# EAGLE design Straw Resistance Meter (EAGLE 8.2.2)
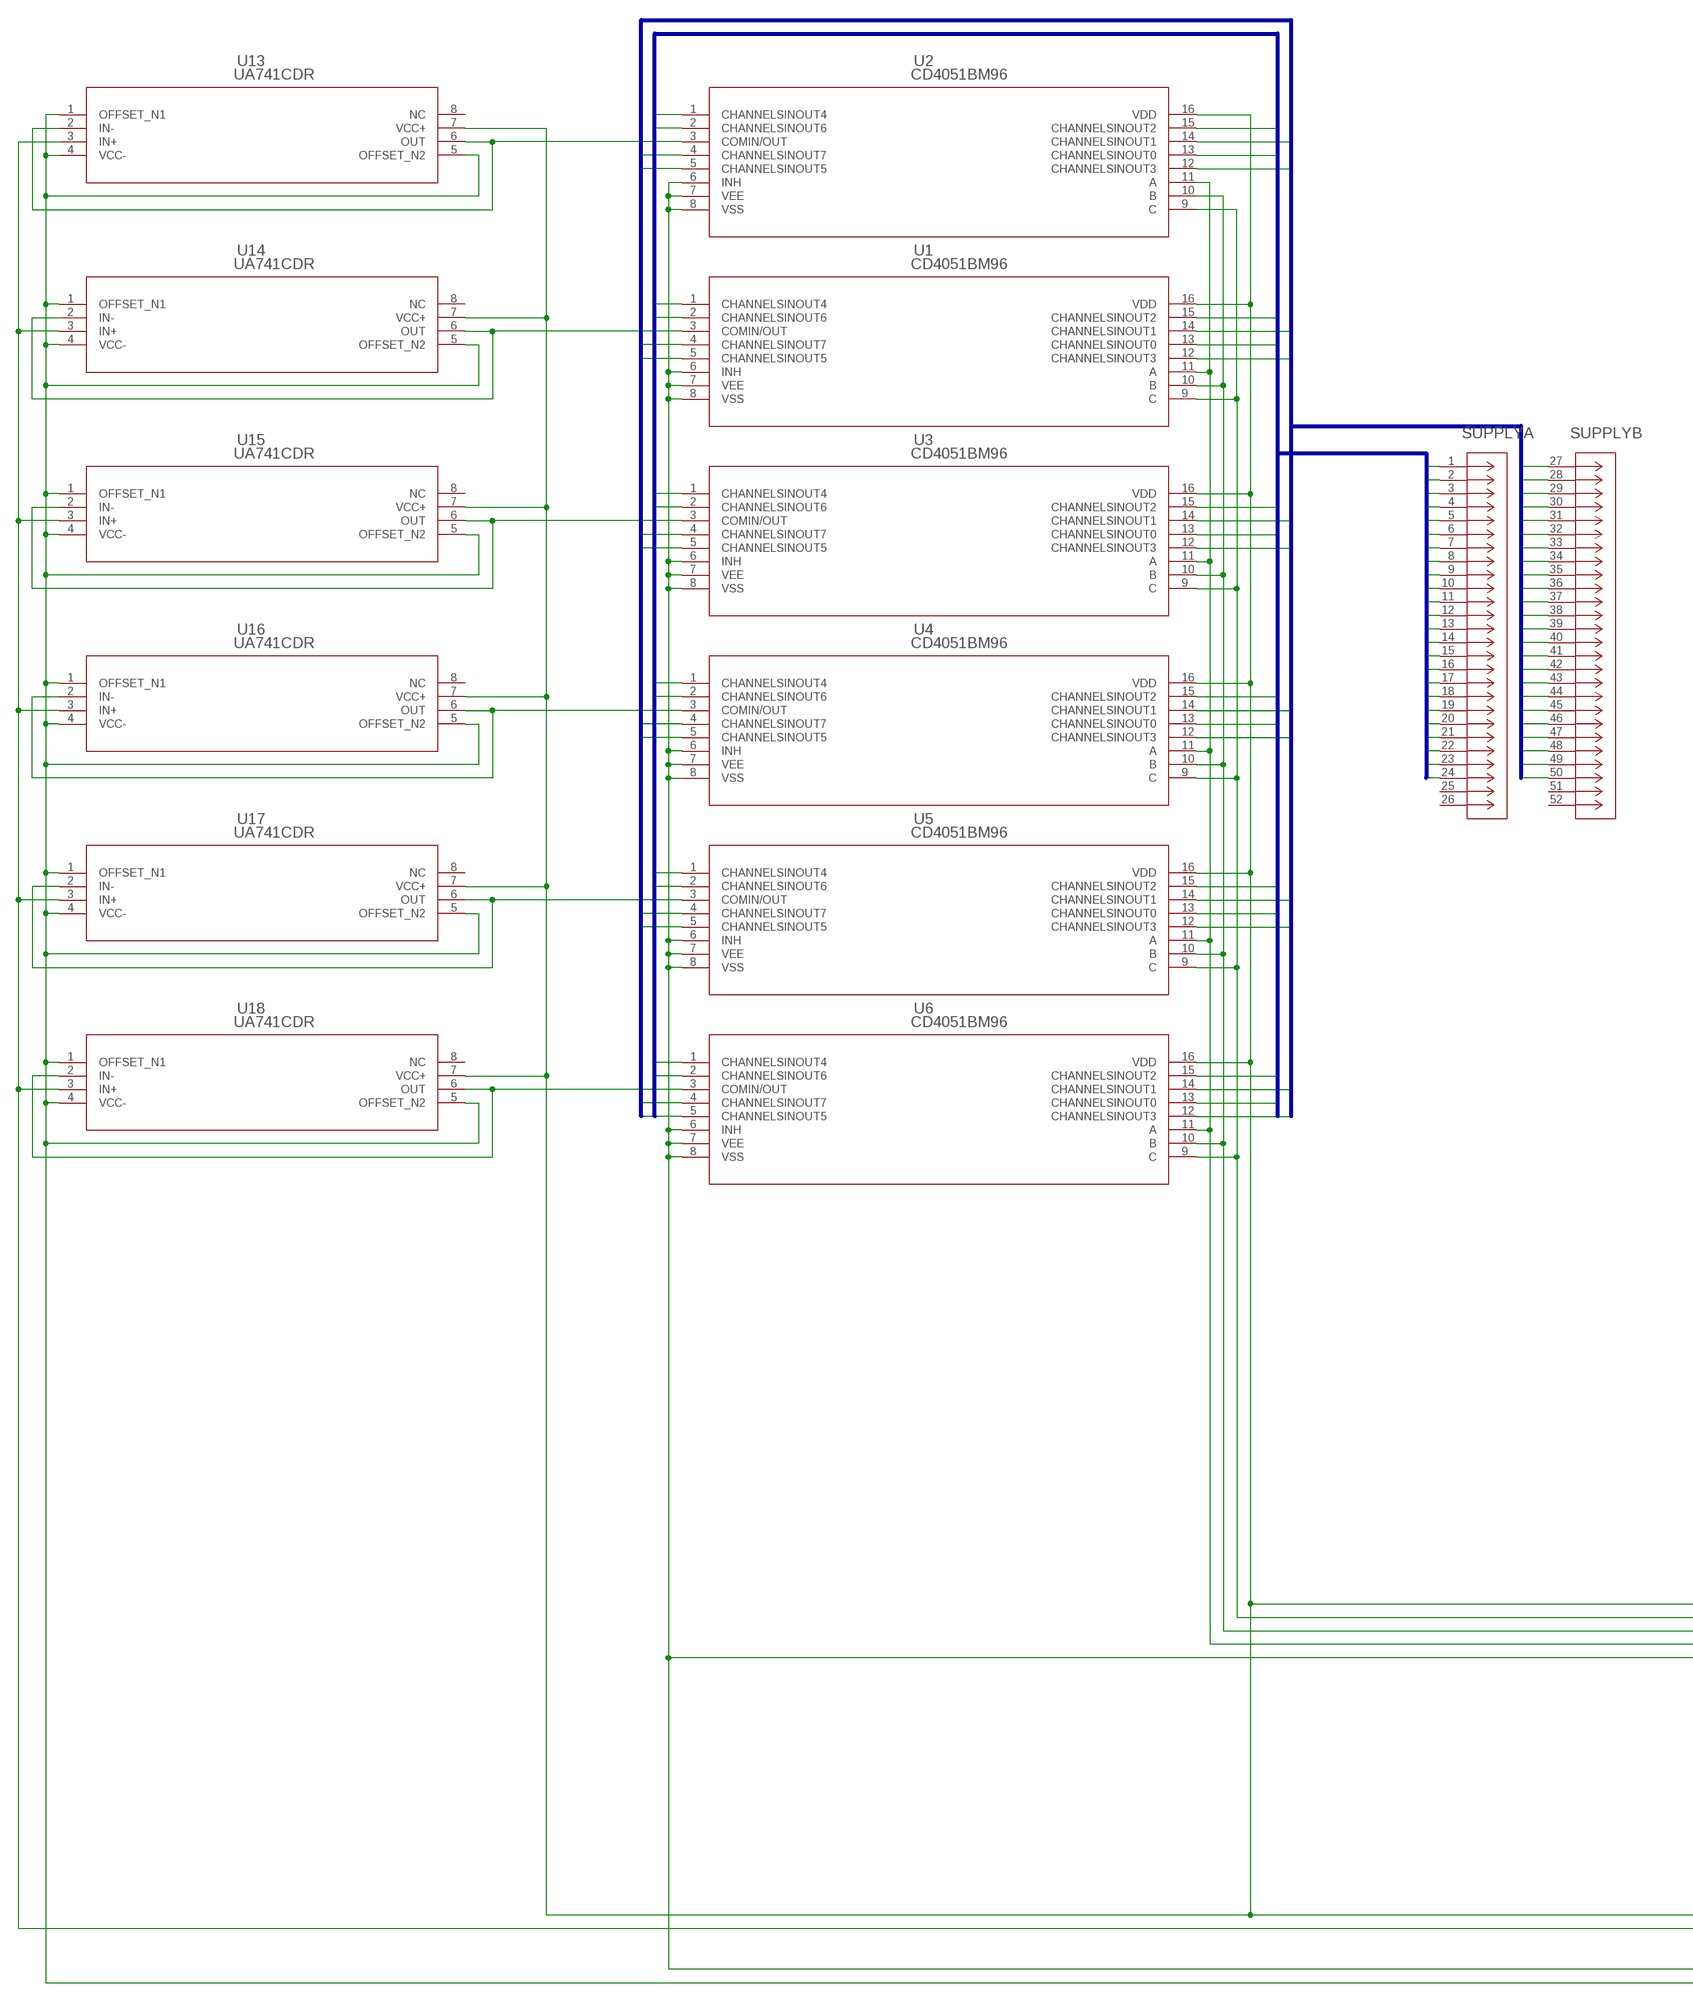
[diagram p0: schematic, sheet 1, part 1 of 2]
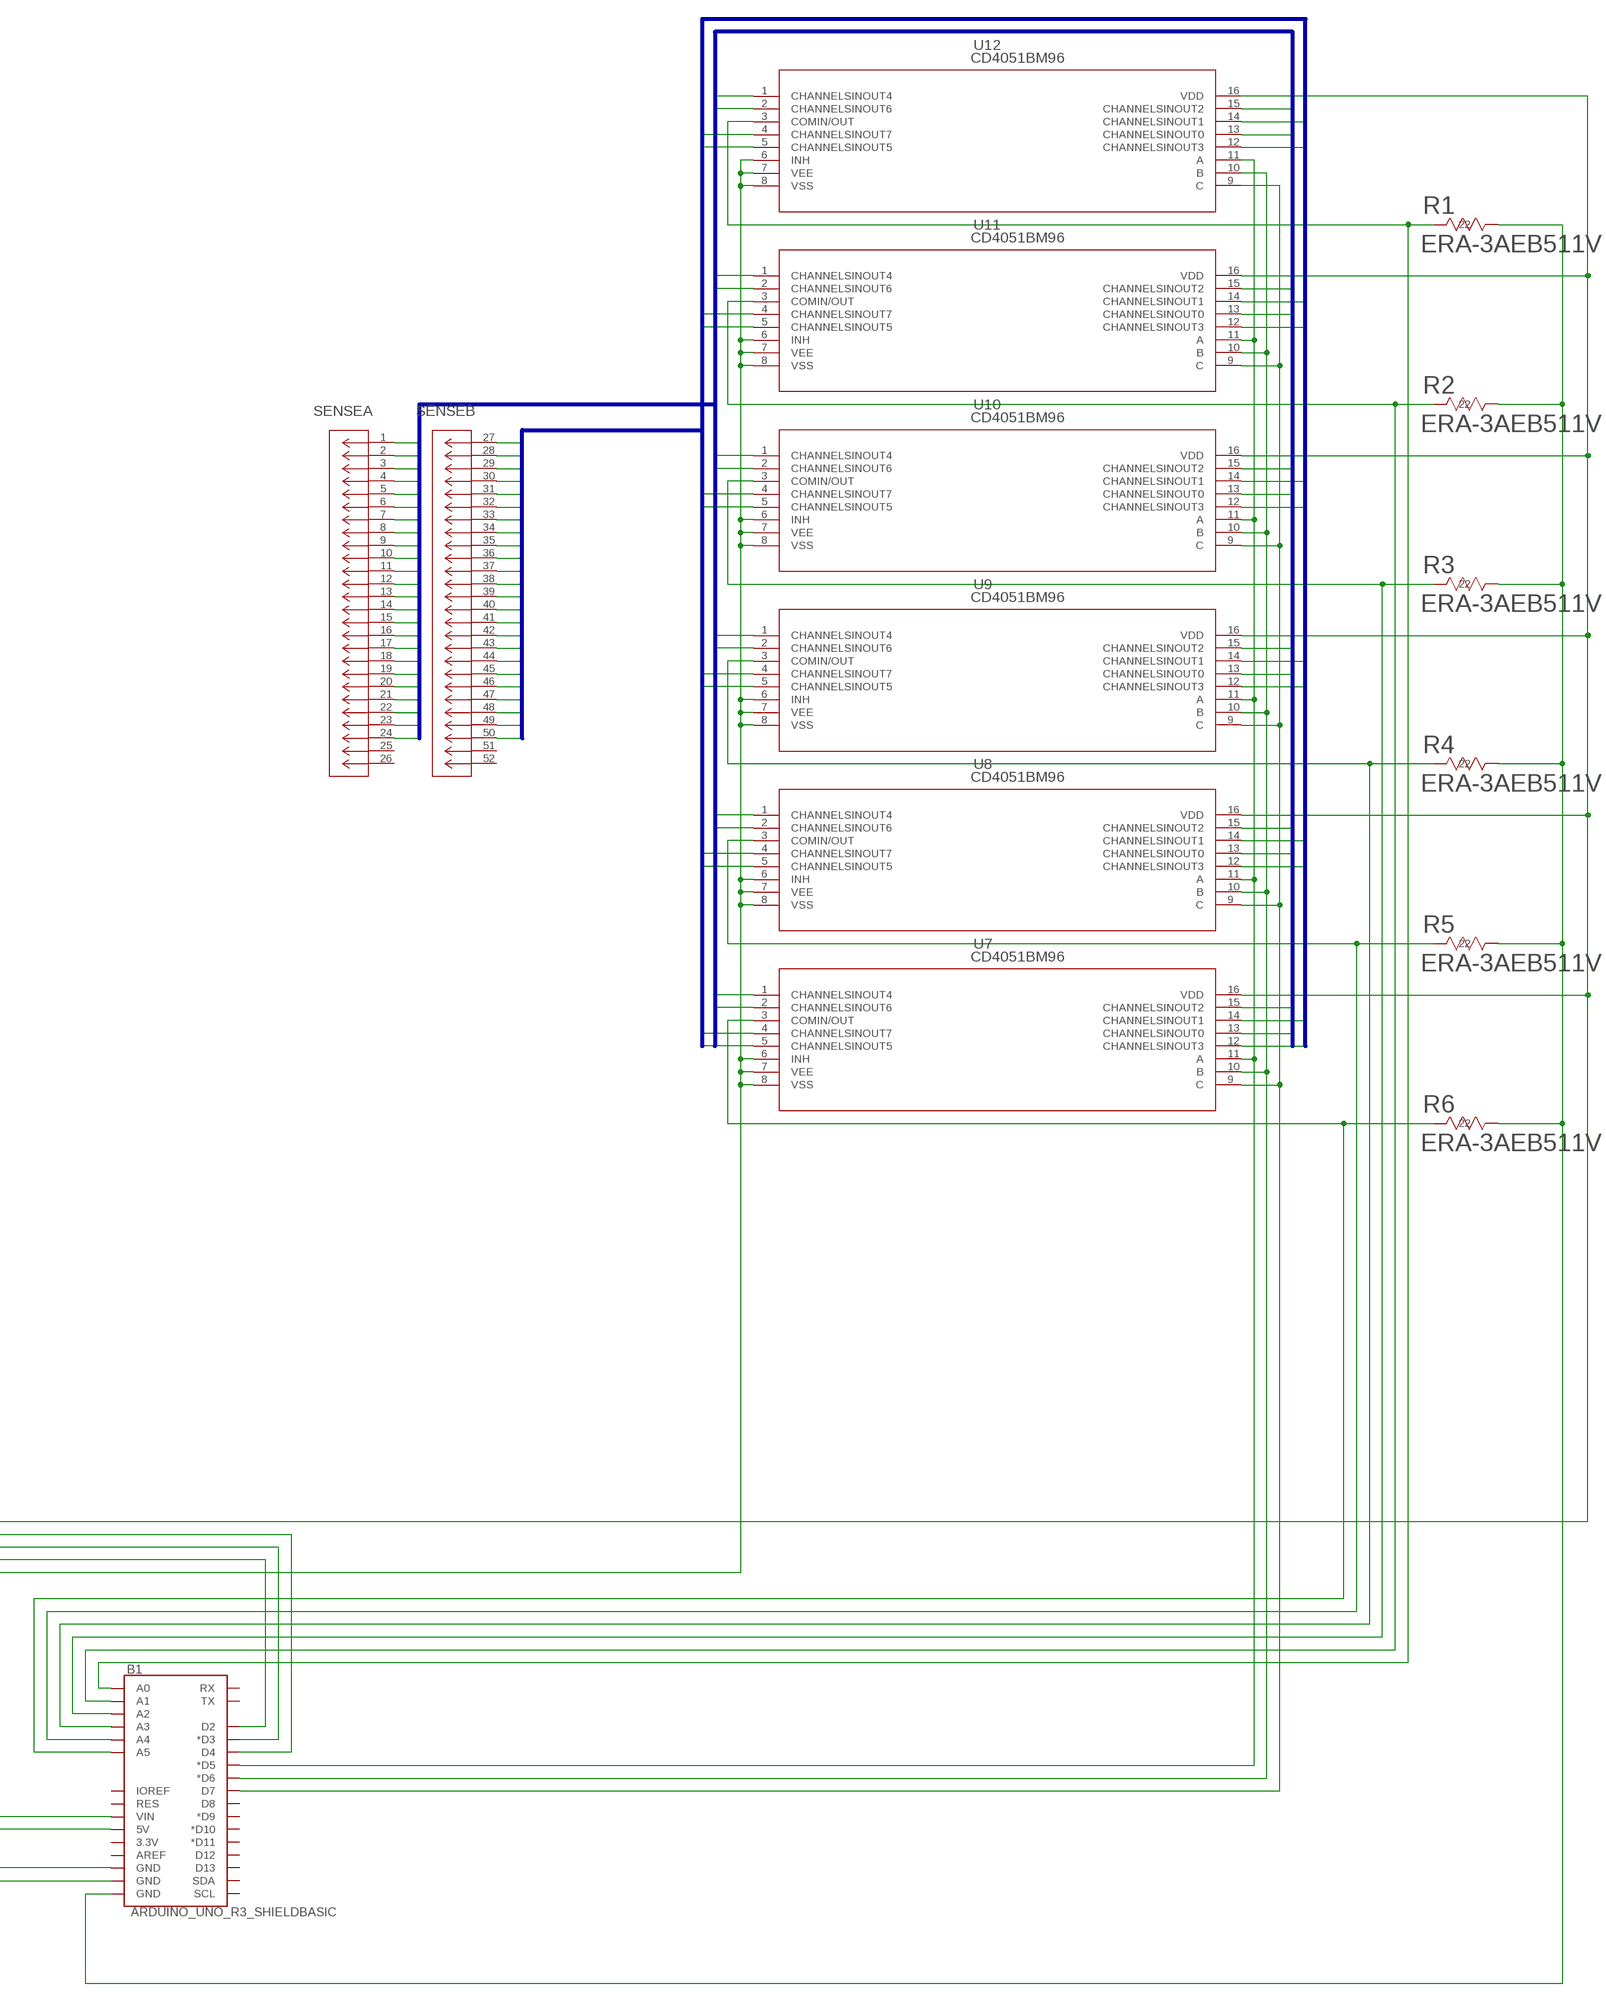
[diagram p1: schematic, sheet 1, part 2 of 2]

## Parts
B1  ARDUINO_UNO_R3_SHIELDBASIC  [UNO_R3_SHIELD]
R1  ERA-3AEB511V  [RC0603N]
R2  ERA-3AEB511V  [RC0603N]
R3  ERA-3AEB511V  [RC0603N]
R4  ERA-3AEB511V  [RC0603N]
R5  ERA-3AEB511V  [RC0603N]
R6  ERA-3AEB511V  [RC0603N]
SENSE  71918-150LF  [CON50_2X25_USZ_FCI]
SUPPLY  71918-150LF  [CON50_2X25_USZ_FCI]
U1  CD4051BM96  [D16]
U2  CD4051BM96  [D16]
U3  CD4051BM96  [D16]
U4  CD4051BM96  [D16]
U5  CD4051BM96  [D16]
U6  CD4051BM96  [D16]
U7  CD4051BM96  [D16]
U8  CD4051BM96  [D16]
U9  CD4051BM96  [D16]
U10  CD4051BM96  [D16]
U11  CD4051BM96  [D16]
U12  CD4051BM96  [D16]
U13  UA741CDR  [D8]
U14  UA741CDR  [D8]
U15  UA741CDR  [D8]
U16  UA741CDR  [D8]
U17  UA741CDR  [D8]
U18  UA741CDR  [D8]

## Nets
INNER_SENSE_BUS0: SENSE.1 U12.13(CHANNELSINOUT0)
INNER_SENSE_BUS1: SENSE.2 U12.15(CHANNELSINOUT2)
INNER_SENSE_BUS2: SENSE.3 U12.1(CHANNELSINOUT4)
INNER_SENSE_BUS3: SENSE.4 U12.2(CHANNELSINOUT6)
INNER_SENSE_BUS4: SENSE.5 U11.13(CHANNELSINOUT0)
INNER_SENSE_BUS5: SENSE.6 U11.15(CHANNELSINOUT2)
INNER_SENSE_BUS6: SENSE.7 U11.1(CHANNELSINOUT4)
INNER_SENSE_BUS7: SENSE.8 U11.2(CHANNELSINOUT6)
INNER_SENSE_BUS8: SENSE.9 U10.13(CHANNELSINOUT0)
INNER_SENSE_BUS9: SENSE.10 U10.15(CHANNELSINOUT2)
INNER_SENSE_BUS10: SENSE.11 U10.1(CHANNELSINOUT4)
INNER_SENSE_BUS11: SENSE.12 U10.2(CHANNELSINOUT6)
INNER_SENSE_BUS12: SENSE.13 U9.13(CHANNELSINOUT0)
INNER_SENSE_BUS13: SENSE.14 U9.15(CHANNELSINOUT2)
INNER_SENSE_BUS14: SENSE.15 U9.1(CHANNELSINOUT4)
INNER_SENSE_BUS15: SENSE.16 U9.2(CHANNELSINOUT6)
INNER_SENSE_BUS16: SENSE.17 U8.13(CHANNELSINOUT0)
INNER_SENSE_BUS17: SENSE.18 U8.15(CHANNELSINOUT2)
INNER_SENSE_BUS18: SENSE.19 U8.1(CHANNELSINOUT4)
INNER_SENSE_BUS19: SENSE.20 U8.2(CHANNELSINOUT6)
INNER_SENSE_BUS20: SENSE.21 U7.13(CHANNELSINOUT0)
INNER_SENSE_BUS21: SENSE.22 U7.15(CHANNELSINOUT2)
INNER_SENSE_BUS22: SENSE.23 U7.1(CHANNELSINOUT4)
INNER_SENSE_BUS23: SENSE.24 U7.2(CHANNELSINOUT6)
INNER_SUPPLY_BUS0: SUPPLY.1 U2.13(CHANNELSINOUT0)
INNER_SUPPLY_BUS1: SUPPLY.2 U2.15(CHANNELSINOUT2)
INNER_SUPPLY_BUS2: SUPPLY.3 U2.1(CHANNELSINOUT4)
INNER_SUPPLY_BUS3: SUPPLY.4 U2.2(CHANNELSINOUT6)
INNER_SUPPLY_BUS4: SUPPLY.5 U1.13(CHANNELSINOUT0)
INNER_SUPPLY_BUS5: SUPPLY.6 U1.15(CHANNELSINOUT2)
INNER_SUPPLY_BUS6: SUPPLY.7 U1.1(CHANNELSINOUT4)
INNER_SUPPLY_BUS7: SUPPLY.8 U1.2(CHANNELSINOUT6)
INNER_SUPPLY_BUS8: SUPPLY.9 U3.13(CHANNELSINOUT0)
INNER_SUPPLY_BUS9: SUPPLY.10 U3.15(CHANNELSINOUT2)
INNER_SUPPLY_BUS10: SUPPLY.11 U3.1(CHANNELSINOUT4)
INNER_SUPPLY_BUS11: SUPPLY.12 U3.2(CHANNELSINOUT6)
INNER_SUPPLY_BUS12: SUPPLY.13 U4.13(CHANNELSINOUT0)
INNER_SUPPLY_BUS13: SUPPLY.14 U4.15(CHANNELSINOUT2)
INNER_SUPPLY_BUS14: SUPPLY.15 U4.1(CHANNELSINOUT4)
INNER_SUPPLY_BUS15: SUPPLY.16 U4.2(CHANNELSINOUT6)
INNER_SUPPLY_BUS16: SUPPLY.17 U5.13(CHANNELSINOUT0)
INNER_SUPPLY_BUS17: SUPPLY.18 U5.15(CHANNELSINOUT2)
INNER_SUPPLY_BUS18: SUPPLY.19 U5.1(CHANNELSINOUT4)
INNER_SUPPLY_BUS19: SUPPLY.20 U5.2(CHANNELSINOUT6)
INNER_SUPPLY_BUS20: SUPPLY.21 U6.13(CHANNELSINOUT0)
INNER_SUPPLY_BUS21: SUPPLY.22 U6.15(CHANNELSINOUT2)
INNER_SUPPLY_BUS22: SUPPLY.23 U6.1(CHANNELSINOUT4)
INNER_SUPPLY_BUS23: SUPPLY.24 U6.2(CHANNELSINOUT6)
N$1 [Power]: B1.GND@2(GND) U1.6(INH) U1.7(VEE) U1.8(VSS) U2.6(INH) U2.7(VEE) U2.8(VSS) U3.6(INH) U3.7(VEE) U3.8(VSS) U4.6(INH) U4.7(VEE) U4.8(VSS) U5.6(INH) U5.7(VEE) U5.8(VSS) U6.6(INH) U6.7(VEE) U6.8(VSS) U7.6(INH) U7.7(VEE) U7.8(VSS) U8.6(INH) U8.7(VEE) U8.8(VSS) U9.6(INH) U9.7(VEE) U9.8(VSS) U10.6(INH) U10.7(VEE) U10.8(VSS) U11.6(INH) U11.7(VEE) U11.8(VSS) U12.6(INH) U12.7(VEE) U12.8(VSS)
N$2: U2.3(COMIN/OUT) U13.2(IN-) U13.6(OUT)
N$3 [Power]: B1.GND@1(GND) U13.1(OFFSET_N1) U13.4(VCC-) U13.5(OFFSET_N2) U14.1(OFFSET_N1) U14.4(VCC-) U14.5(OFFSET_N2) U15.1(OFFSET_N1) U15.4(VCC-) U15.5(OFFSET_N2) U16.1(OFFSET_N1) U16.4(VCC-) U16.5(OFFSET_N2) U17.1(OFFSET_N1) U17.4(VCC-) U17.5(OFFSET_N2) U18.1(OFFSET_N1) U18.4(VCC-) U18.5(OFFSET_N2)
N$4 [Power]: B1.VIN U1.16(VDD) U2.16(VDD) U3.16(VDD) U4.16(VDD) U5.16(VDD) U6.16(VDD) U7.16(VDD) U8.16(VDD) U9.16(VDD) U10.16(VDD) U11.16(VDD) U12.16(VDD) U13.7(VCC+) U14.7(VCC+) U15.7(VCC+) U16.7(VCC+) U17.7(VCC+) U18.7(VCC+)
N$5 [Power]: B1.5V U13.3(IN+) U14.3(IN+) U15.3(IN+) U16.3(IN+) U17.3(IN+) U18.3(IN+)
N$6: B1.D4 U1.9(C) U2.9(C) U3.9(C) U4.9(C) U5.9(C) U6.9(C)
N$7: U1.3(COMIN/OUT) U14.2(IN-) U14.6(OUT)
N$8: B1.D3(*D3) U1.10(B) U2.10(B) U3.10(B) U4.10(B) U5.10(B) U6.10(B)
N$9: B1.D2 U1.11(A) U2.11(A) U3.11(A) U4.11(A) U5.11(A) U6.11(A)
N$10: U3.3(COMIN/OUT) U15.2(IN-) U15.6(OUT)
N$11: B1.D5(*D5) U7.11(A) U8.11(A) U9.11(A) U10.11(A) U11.11(A) U12.11(A)
N$12: B1.D6(*D6) U7.10(B) U8.10(B) U9.10(B) U10.10(B) U11.10(B) U12.10(B)
N$13: U4.3(COMIN/OUT) U16.2(IN-) U16.6(OUT)
N$14: B1.D7 U7.9(C) U8.9(C) U9.9(C) U10.9(C) U11.9(C) U12.9(C)
N$15: B1.A0 R1.2 U12.3(COMIN/OUT)
N$16: U5.3(COMIN/OUT) U17.2(IN-) U17.6(OUT)
N$17: B1.A1 R2.2 U11.3(COMIN/OUT)
N$18: B1.A3 R4.2 U9.3(COMIN/OUT)
N$19: U6.3(COMIN/OUT) U18.2(IN-) U18.6(OUT)
N$20: B1.A4 R5.2 U8.3(COMIN/OUT)
N$21 [Power]: B1.GND@0(GND) R1.1 R2.1 R3.1 R4.1 R5.1 R6.1
N$22: B1.A5 R6.2 U7.3(COMIN/OUT)
N$23: B1.A2 R3.2 U10.3(COMIN/OUT)
OUTER_SENSE_BUS0: SENSE.27 U12.14(CHANNELSINOUT1)
OUTER_SENSE_BUS1: SENSE.28 U12.12(CHANNELSINOUT3)
OUTER_SENSE_BUS2: SENSE.29 U12.5(CHANNELSINOUT5)
OUTER_SENSE_BUS3: SENSE.30 U12.4(CHANNELSINOUT7)
OUTER_SENSE_BUS4: SENSE.31 U11.14(CHANNELSINOUT1)
OUTER_SENSE_BUS5: SENSE.32 U11.12(CHANNELSINOUT3)
OUTER_SENSE_BUS6: SENSE.33 U11.5(CHANNELSINOUT5)
OUTER_SENSE_BUS7: SENSE.34 U11.4(CHANNELSINOUT7)
OUTER_SENSE_BUS8: SENSE.35 U10.14(CHANNELSINOUT1)
OUTER_SENSE_BUS9: SENSE.36 U10.12(CHANNELSINOUT3)
OUTER_SENSE_BUS10: SENSE.37 U10.5(CHANNELSINOUT5)
OUTER_SENSE_BUS11: SENSE.38 U10.4(CHANNELSINOUT7)
OUTER_SENSE_BUS12: SENSE.39 U9.14(CHANNELSINOUT1)
OUTER_SENSE_BUS13: SENSE.40 U9.12(CHANNELSINOUT3)
OUTER_SENSE_BUS14: SENSE.41 U9.5(CHANNELSINOUT5)
OUTER_SENSE_BUS15: SENSE.42 U9.4(CHANNELSINOUT7)
OUTER_SENSE_BUS16: SENSE.43 U8.14(CHANNELSINOUT1)
OUTER_SENSE_BUS17: SENSE.44 U8.12(CHANNELSINOUT3)
OUTER_SENSE_BUS18: SENSE.45 U8.5(CHANNELSINOUT5)
OUTER_SENSE_BUS19: SENSE.46 U8.4(CHANNELSINOUT7)
OUTER_SENSE_BUS20: SENSE.47 U7.14(CHANNELSINOUT1)
OUTER_SENSE_BUS21: SENSE.48 U7.12(CHANNELSINOUT3)
OUTER_SENSE_BUS22: SENSE.49 U7.5(CHANNELSINOUT5)
OUTER_SENSE_BUS23: SENSE.50 U7.4(CHANNELSINOUT7)
OUTER_SUPPLY_BUS0: SUPPLY.27 U2.14(CHANNELSINOUT1)
OUTER_SUPPLY_BUS1: SUPPLY.28 U2.12(CHANNELSINOUT3)
OUTER_SUPPLY_BUS2: SUPPLY.29 U2.5(CHANNELSINOUT5)
OUTER_SUPPLY_BUS3: SUPPLY.30 U2.4(CHANNELSINOUT7)
OUTER_SUPPLY_BUS4: SUPPLY.31 U1.14(CHANNELSINOUT1)
OUTER_SUPPLY_BUS5: SUPPLY.32 U1.12(CHANNELSINOUT3)
OUTER_SUPPLY_BUS6: SUPPLY.33 U1.5(CHANNELSINOUT5)
OUTER_SUPPLY_BUS7: SUPPLY.34 U1.4(CHANNELSINOUT7)
OUTER_SUPPLY_BUS8: SUPPLY.35 U3.14(CHANNELSINOUT1)
OUTER_SUPPLY_BUS9: SUPPLY.36 U3.12(CHANNELSINOUT3)
OUTER_SUPPLY_BUS10: SUPPLY.37 U3.5(CHANNELSINOUT5)
OUTER_SUPPLY_BUS11: SUPPLY.38 U3.4(CHANNELSINOUT7)
OUTER_SUPPLY_BUS12: SUPPLY.39 U4.14(CHANNELSINOUT1)
OUTER_SUPPLY_BUS13: SUPPLY.40 U4.12(CHANNELSINOUT3)
OUTER_SUPPLY_BUS14: SUPPLY.41 U4.5(CHANNELSINOUT5)
OUTER_SUPPLY_BUS15: SUPPLY.42 U4.4(CHANNELSINOUT7)
OUTER_SUPPLY_BUS16: SUPPLY.43 U5.14(CHANNELSINOUT1)
OUTER_SUPPLY_BUS17: SUPPLY.44 U5.12(CHANNELSINOUT3)
OUTER_SUPPLY_BUS18: SUPPLY.45 U5.5(CHANNELSINOUT5)
OUTER_SUPPLY_BUS19: SUPPLY.46 U5.4(CHANNELSINOUT7)
OUTER_SUPPLY_BUS20: SUPPLY.47 U6.14(CHANNELSINOUT1)
OUTER_SUPPLY_BUS21: SUPPLY.48 U6.12(CHANNELSINOUT3)
OUTER_SUPPLY_BUS22: SUPPLY.49 U6.5(CHANNELSINOUT5)
OUTER_SUPPLY_BUS23: SUPPLY.50 U6.4(CHANNELSINOUT7)
Unconnected: B1.3.3V B1.AREF B1.D8 B1.D9(*D9) B1.D10(*D10) B1.D11(*D11) B1.D12 B1.D13 B1.IOREF B1.RES B1.RX B1.SCL B1.SDA B1.TX SENSE.25 SENSE.26 SENSE.51 SENSE.52 SUPPLY.25 SUPPLY.26 SUPPLY.51 SUPPLY.52 U13.8(NC) U14.8(NC) U15.8(NC) U16.8(NC) U17.8(NC) U18.8(NC)

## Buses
INNER_SUPPLY_BUS[0..23]
OUTER_SUPPLY_BUS[0..23]
INNER_SENSE_BUS[0..23]
OUTER_SENSE_BUS[0..23]

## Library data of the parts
B1 = SparkFun-Boards:ARDUINO_UNO_R3_SHIELD: Arduino R3 Shield Footprint Shield form compatible with the Arduino Uno R3. SparkFun Products: MG2639 Cellular Shield MIDI Shield R3 Stackable Headers Kit
R1-R6 = P510DBCT-ND:ERA-3AEB511V; MANUFACTURER_PART_NUMBER: ERA3AEB511V; VENDOR: Panasonic
SENSE SUPPLY = 609-1759-ND:71918-150LF; MANUFACTURER_PART_NUMBER: 71918150LF; VENDOR: FCI
U1-U12 = 296-14271-1-ND:CD4051BM96; MANUFACTURER_PART_NUMBER: CD4051BM96; VENDOR: Texas Instruments
U13-U18 = opamp_ti:UA741CDR; MANUFACTURER_PART_NUMBER: UA741CDR; VENDOR: Texas Instruments

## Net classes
0 default: width 0.254 mm, drill 0.3 mm, clearance 0.152 mm
1 Power: width 0.61 mm, drill 0.3 mm, clearance 0.152 mm

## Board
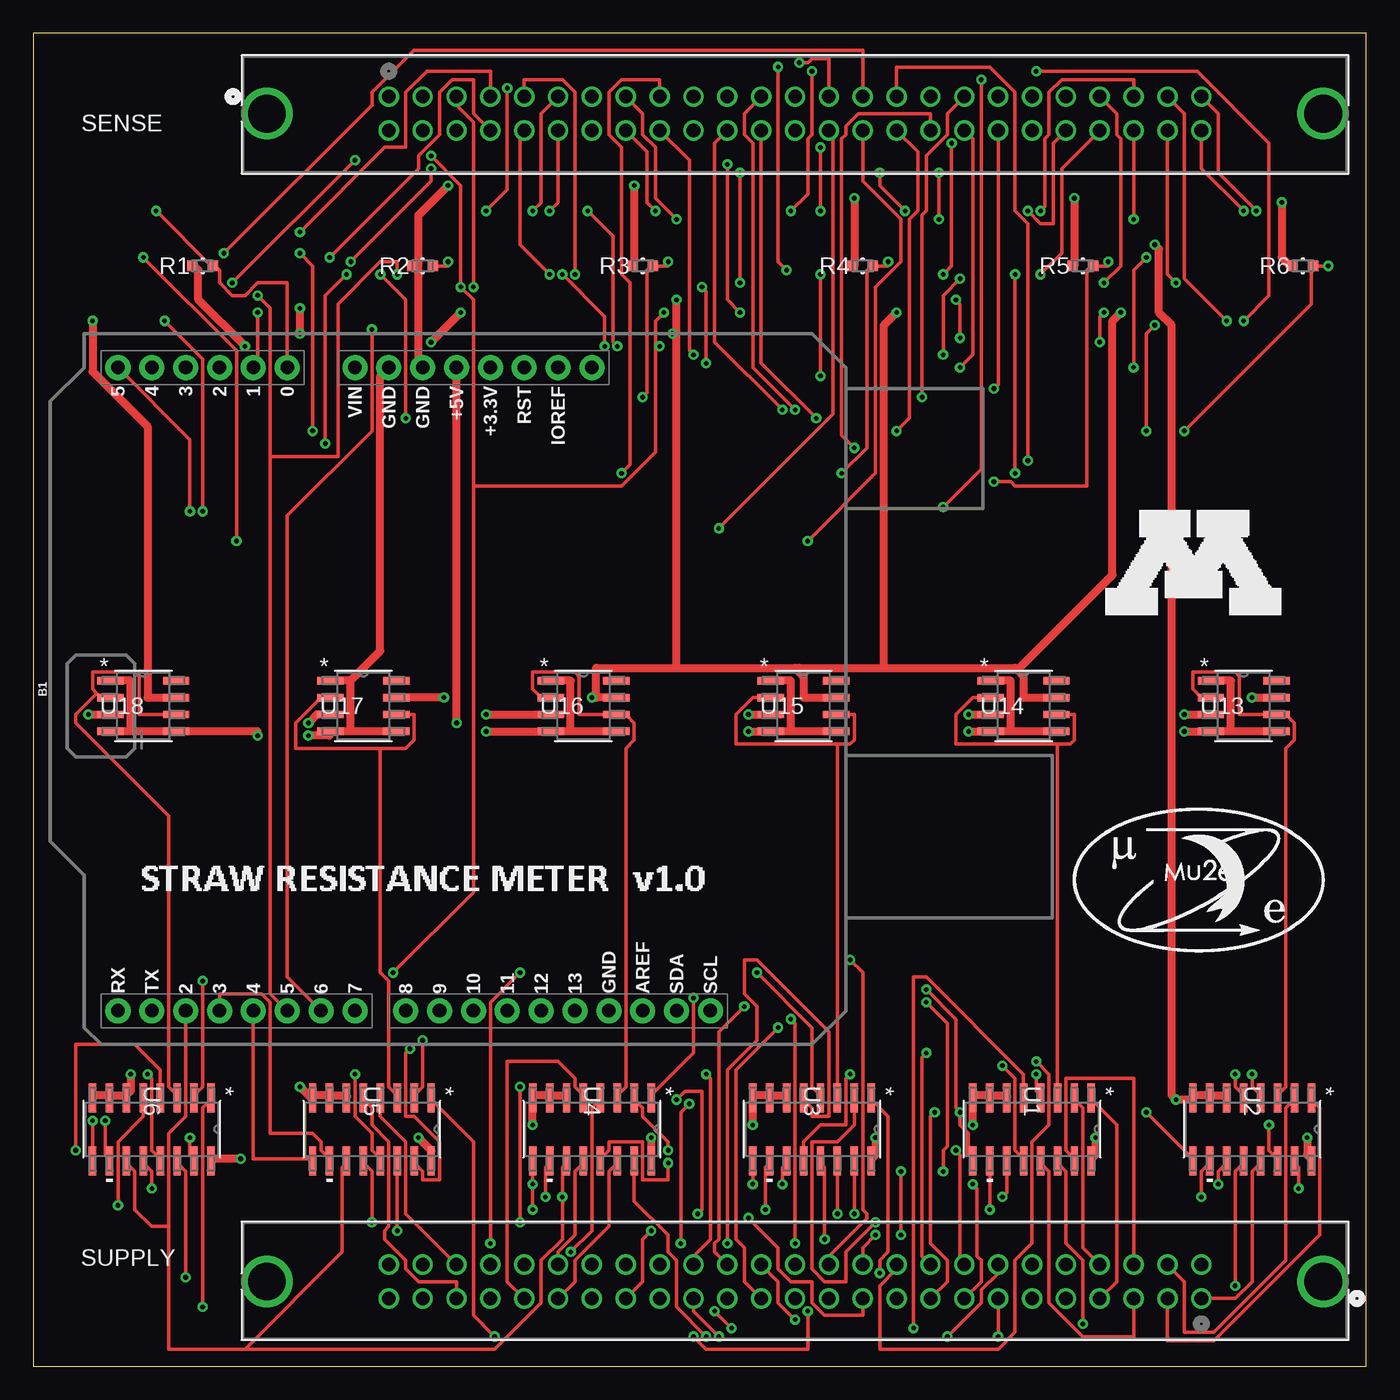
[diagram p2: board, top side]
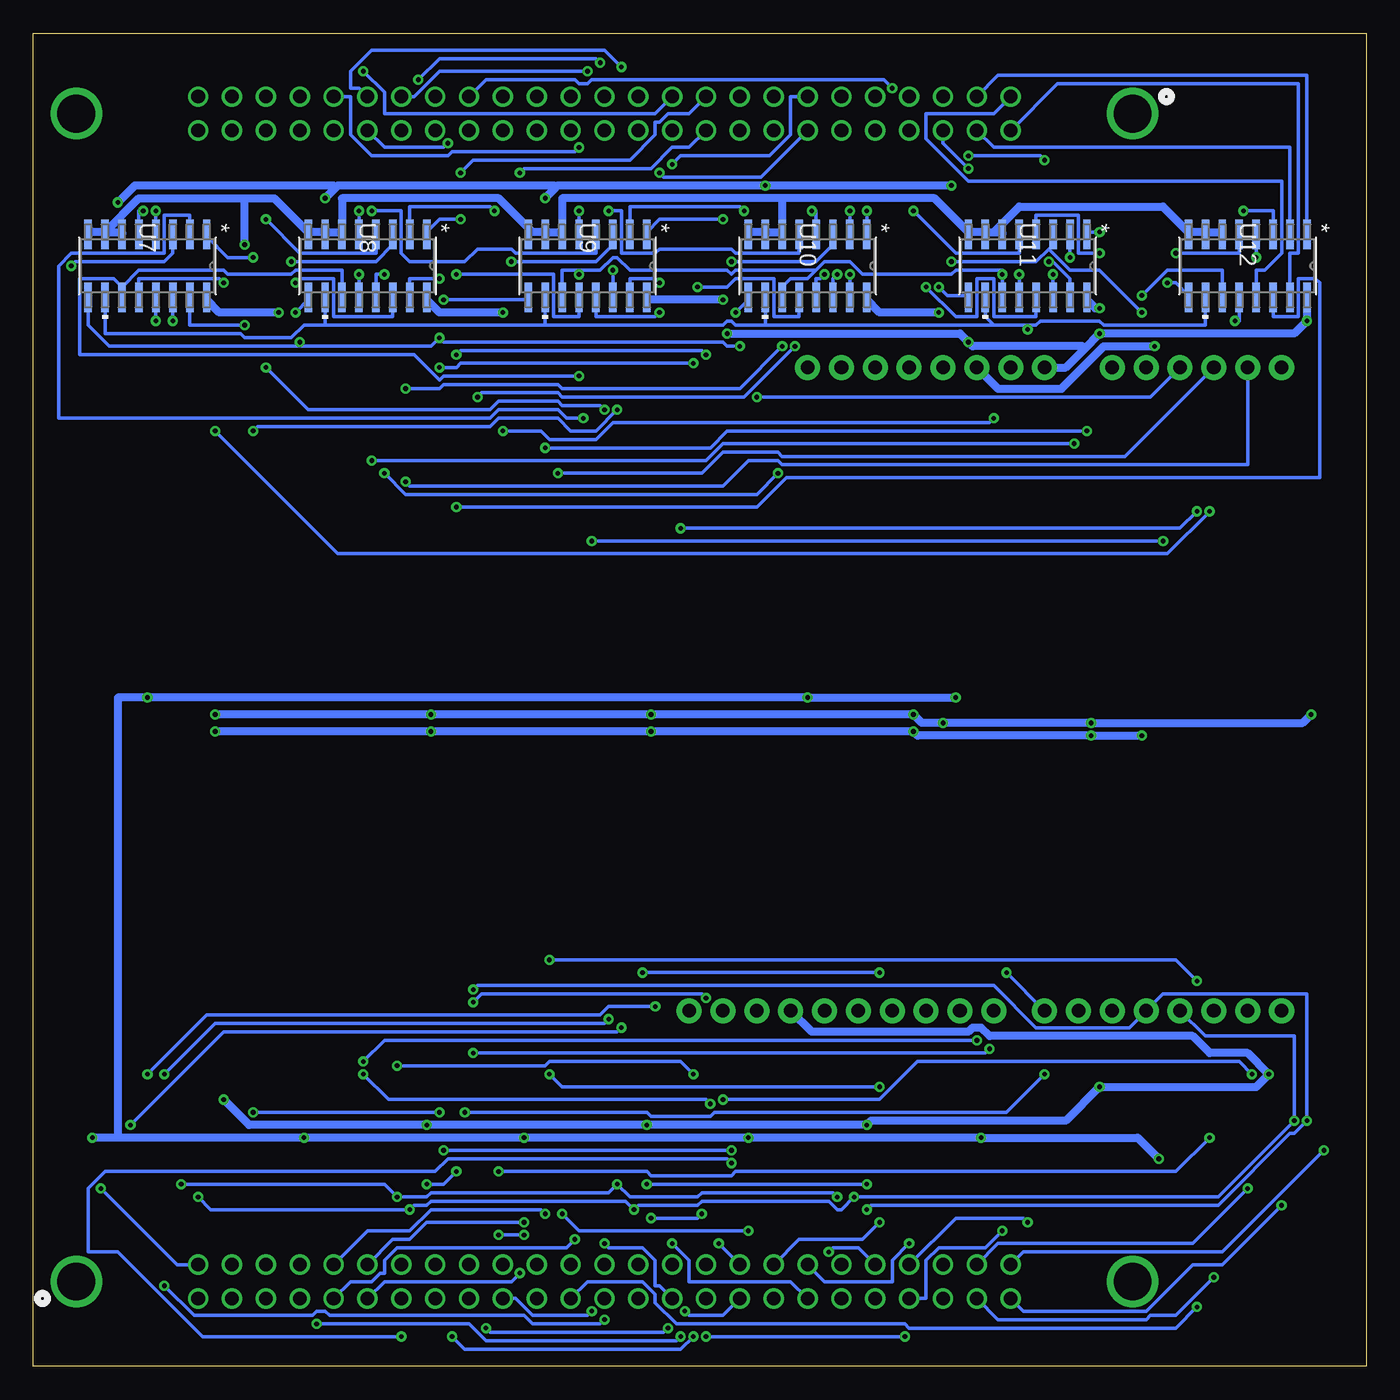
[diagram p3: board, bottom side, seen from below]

Size 100 x 100 mm. Coordinates in mm from the lower left corner, seen from the top.
Outline: 0,0 100,0 100,100 0,100 0,0
Copper layers (1*16): Top 0.035mm / dielectric 1.5mm / Bottom 0.035mm
Design rules "default": minimum track width 6mil, minimum drill 0.35mm, track to track 6mil, track to pad 6mil, pad to pad 6mil, via to via 6mil, smd to smd 6mil, copper to edge 40mil, drill to drill 6mil, minimum pad ring 10mil, minimum via ring 8mil, stop-mask expansion 4mil, vias tented up to drill 0mil, thermal gap 10mil

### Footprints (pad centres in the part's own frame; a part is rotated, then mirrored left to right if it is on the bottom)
UNO_R3_SHIELD = drill 1.016 pad 1.88: 3.3V 24.13,-2.54; 5V 24.13,0; A0 24.13,12.7; A1 24.13,15.24; A2 24.13,17.78; A3 24.13,20.32; A4 24.13,22.86; A5 24.13,25.4; AREF -24.13,-13.97; D2 -24.13,20.32; D3 -24.13,17.78; D4 -24.13,15.24; D5 -24.13,12.7; D6 -24.13,10.16; D7 -24.13,7.62; D8 -24.13,3.81; D9 -24.13,1.27; D10 -24.13,-1.27; D11 -24.13,-3.81; D12 -24.13,-6.35; D13 -24.13,-8.89; GND@0 24.13,2.54; GND@1 24.13,5.08; GND@2 -24.13,-11.43; IOREF 24.13,-7.62; NC 24.13,-10.16; RES 24.13,-5.08; RX -24.13,25.4; SCL -24.13,-19.05; SDA -24.13,-16.51; TX -24.13,22.86; VIN 24.13,7.62
RC0603N = smd 0.756 x 0.8: 1 -0.778,0; 2 0.778,0
CON50_2X25_USZ_FCI = drill 1.016 pad 1.524: 1 -60.96,2.54; 2 -60.96,0; 3 -58.42,2.54; 4 -58.42,0; 5 -55.88,2.54; 6 -55.88,0; 7 -53.34,2.54; 8 -53.34,0; 9 -50.8,2.54; 10 -50.8,0; 11 -48.26,2.54; 12 -48.26,0; 13 -45.72,2.54; 14 -45.72,0; 15 -43.18,2.54; 16 -43.18,0; 17 -40.64,2.54; 18 -40.64,0; 19 -38.1,2.54; 20 -38.1,0; 21 -35.56,2.54; 22 -35.56,0; 23 -33.02,2.54; 24 -33.02,0; 25 -30.48,2.54; 26 -30.48,0; 27 -27.94,2.54; 28 -27.94,0; 29 -25.4,2.54; 30 -25.4,0; 31 -22.86,2.54; 32 -22.86,0; 33 -20.32,2.54; 34 -20.32,0; 35 -17.78,2.54; 36 -17.78,0; 37 -15.24,2.54; 38 -15.24,0; 39 -12.7,2.54; 40 -12.7,0; 41 -10.16,2.54; 42 -10.16,0; 43 -7.62,2.54; 44 -7.62,0; 45 -5.08,2.54; 46 -5.08,0; 47 -2.54,2.54; 48 -2.54,0; 49 0,2.54; 50 0,0 | drill 2.845 pad 3.353: 51 -70.104,1.27; 52 9.144,1.27
D16 = smd 2.184 x 0.559: 1 -2.362,4.445; 2 -2.362,3.175; 3 -2.362,1.905; 4 -2.362,0.635; 5 -2.362,-0.635; 6 -2.362,-1.905; 7 -2.362,-3.175; 8 -2.362,-4.445; 9 2.362,-4.445; 10 2.362,-3.175; 11 2.362,-1.905; 12 2.362,-0.635; 13 2.362,0.635; 14 2.362,1.905; 15 2.362,3.175; 16 2.362,4.445
D8 = smd 1.981 x 0.559: 1 -2.464,1.905; 2 -2.464,0.635; 3 -2.464,-0.635; 4 -2.464,-1.905; 5 2.464,-1.905; 6 2.464,-0.635; 7 2.464,0.635; 8 2.464,1.905

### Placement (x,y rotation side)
B1  31.75,50.8 90 top
R1  12.7,82.55 0 top
R2  29.21,82.55 0 top
R3  45.72,82.55 0 top
R4  62.23,82.55 0 top
R5  78.74,82.55 0 top
R6  95.25,82.55 0 top
SENSE  87.63,92.71 0 top
SUPPLY  26.67,7.62 180 top
U1  74.93,17.78 270 top
U2  91.44,17.78 270 top
U3  58.42,17.78 270 top
U4  41.91,17.78 270 top
U5  25.4,17.78 270 top
U6  8.89,17.78 270 top
U7  91.44,82.55 270 bottom
U8  74.93,82.55 270 bottom
U9  58.42,82.55 270 bottom
U10  41.91,82.55 270 bottom
U11  25.4,82.55 270 bottom
U12  8.89,82.55 270 bottom
U13  90.81,49.53 0 top
U14  74.3,49.53 0 top
U15  57.78,49.53 0 top
U16  41.27,49.53 0 top
U17  24.77,49.53 0 top
U18  8.26,49.53 0 top

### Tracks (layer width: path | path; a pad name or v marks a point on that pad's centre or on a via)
INNER_SENSE_BUS0
  Bottom 0.254: U12.13 8.26,82.23 7.62,82.23 6.35,83.5 6.35,88.9 29.84,88.9 33.02,92.08 33.02,93.98 27.94,93.98 SENSE.1
INNER_SENSE_BUS1
  Bottom 0.254: U12.15 5.71,83.5 5.08,83.5 5.08,96.2 23.18,96.2 SENSE.2
INNER_SENSE_BUS2
  Bottom 0.254: U12.1 4.45,96.84 27.62,96.84 SENSE.3
INNER_SENSE_BUS3
  Bottom 0.254: U12.2 5.71,91.44 27.94,91.44 SENSE.4
INNER_SENSE_BUS4  (via drill 0.35)
  Top 0.254: v33.02,80.96 33.02,93.34 31.75,94.61 SENSE.5
  Bottom 0.254: U11.13 24.77,78.74 27.94,78.74 27.94,81.6 29.21,81.6 29.21,78.74 30.8,78.74 v33.02,80.96
INNER_SENSE_BUS5  (via drill 0.35)
  Top 0.254: v23.81,82.87 29.84,88.9 v29.84,89.85
  Bottom 0.254: U11.15 22.23,81.6 23.5,82.87 v23.81,82.87 | v29.84,89.85 31.75,91.76 SENSE.6
INNER_SENSE_BUS6  (via drill 0.35)
  Top 0.254: v20,85.09 26.35,91.44 27.94,91.44 27.94,95.57 29.53,97.16 34.29,97.16 SENSE.7
  Bottom 0.254: v20,85.09 20.95,85.09 U11.1
INNER_SENSE_BUS7  (via drill 0.35)
  Top 0.254: v22.23,83.19 28.89,89.85 28.89,90.81 30.48,92.39 30.48,95.57 31.43,96.52 33.02,96.52 33.02,93.98 SENSE.8
  Bottom 0.254: v22.23,83.19 U11.2
INNER_SENSE_BUS8  (via drill 0.35)
  Top 0.254: v40.64,81.92 40.64,95.57 39.69,96.52 36.83,96.52 SENSE.9
  Bottom 0.254: U10.13 41.27,81.6 40.96,81.6 v40.64,81.92
INNER_SENSE_BUS9  (via drill 0.35)
  Top 0.254: v38.73,81.92 36.51,84.14 36.51,92.39 SENSE.10
  Bottom 0.254: v38.73,81.92 U10.15
INNER_SENSE_BUS10  (via drill 0.35)
  Top 0.254: v37.47,86.68 38.1,87.31 38.1,93.98 SENSE.11
  Bottom 0.254: v37.47,86.68 U10.1
INNER_SENSE_BUS11  (via drill 0.35)
  Top 0.254: v38.73,86.68 39.37,87.31 SENSE.12
  Bottom 0.254: v38.73,86.68 U10.2
INNER_SENSE_BUS12  (via drill 0.35)
  Top 0.254: v53.02,79.06 52.07,80.01 v52.07,90.17
  Bottom 0.254: U9.13 57.78,78.74 53.34,78.74 v53.02,79.06 | v52.07,90.17 51.44,90.81 44.77,90.81 43.18,92.39 43.18,95.25 SENSE.13
INNER_SENSE_BUS13  (via drill 0.35)
  Top 0.254: v53.02,89.53 v53.02,81.28
  Bottom 0.254: U9.15 55.24,81.6 53.34,81.6 v53.02,81.28 | v53.02,89.53 52.7,89.22 45.4,89.22 SENSE.14
INNER_SENSE_BUS14  (via drill 0.35)
  Top 0.254: v48.26,86.04 46.67,87.63 46.67,91.44 45.72,92.39 45.72,93.98 SENSE.15
  Bottom 0.254: v48.26,86.04 53.02,86.04 53.98,85.09 U9.1
INNER_SENSE_BUS15  (via drill 0.35)
  Top 0.254: v46.67,86.68 46.04,87.31 46.04,91.12 SENSE.16
  Bottom 0.254: U9.2 55.24,87 46.99,87 v46.67,86.68
INNER_SENSE_BUS16  (via drill 0.35)
  Top 0.254: v73.66,66.99 v73.66,81.92 | v44.13,66.99 44.77,67.63 44.77,81.28 44.13,81.92 44.13,91.44 43.18,92.39 43.18,95.57 44.13,96.52 46.99,96.52 SENSE.17
  Bottom 0.254: U8.13 74.3,81.92 v73.66,81.92 | v73.66,66.99 72.07,65.41 45.72,65.41 v44.13,66.99
INNER_SENSE_BUS17  (via drill 0.35)
  Top 0.254: v69.53,81.6 68.26,80.33 v68.26,75.88 | v49.53,75.88 49.21,76.2 49.21,90.49 SENSE.18
  Bottom 0.254: U8.15 71.75,81.6 v69.53,81.6 | v68.26,75.88 67.94,76.2 49.85,76.2 v49.53,75.88
INNER_SENSE_BUS18  (via drill 0.35)
  Top 0.254: v67.94,89.53 v67.94,86.04
  Bottom 0.254: v67.94,86.04 69.53,86.04 70.48,85.09 U8.1 | v67.94,89.53 66.99,90.49 55.24,90.49 53.34,92.39 53.34,93.34 53.02,93.34 52.39,93.98 50.8,93.98 SENSE.19
INNER_SENSE_BUS19  (via drill 0.35)
  Top 0.254: v65.41,86.68 63.5,88.58 v63.5,89.53
  Bottom 0.254: U8.2 71.75,87 65.72,87 v65.41,86.68 | v63.5,89.53 63.18,89.85 53.66,89.85 52.07,91.44 50.8,91.44 SENSE.20
INNER_SENSE_BUS20  (via drill 0.35)
  Top 0.254: v90.81,78.42 92.71,80.33 92.71,91.76 87.31,97.16 v75.25,97.16
  Bottom 0.254: v90.81,78.42 U7.13 | v75.25,97.16 73.66,95.57 73.66,93.98 53.34,93.98 SENSE.21
INNER_SENSE_BUS21  (via drill 0.35)
  Top 0.254: v84.14,78.11 83.5,77.47 v83.5,70.17 | v56.2,71.75 51.12,76.83 51.12,91.76 SENSE.22
  Bottom 0.254: U7.15 88.27,78.11 v84.14,78.11 | v83.5,70.17 83.19,70.48 65.72,70.48 65.09,71.12 60.64,71.12 59.69,70.17 57.78,70.17 v56.2,71.75
INNER_SENSE_BUS22  (via drill 0.35)
  Top 0.254: v83.5,83.19 82.55,82.23 v82.55,74.93 | v57.15,71.75 53.98,74.93 53.98,91.76 53.34,92.39 53.34,93.98 SENSE.23
  Bottom 0.254: v83.5,83.19 85.41,83.19 87,84.77 U7.1 | v82.55,74.93 79.38,71.75 65.72,71.75 65.09,72.39 60.64,72.39 60.33,72.07 57.47,72.07 v57.15,71.75
INNER_SENSE_BUS23  (via drill 0.35)
  Top 0.254: v58.74,71.12 54.61,75.25 SENSE.24
  Bottom 0.254: U7.2 88.27,86.36 90.17,86.36 90.17,83.5 97.16,83.5 98.11,82.55 98.11,71.12 65.72,71.12 65.09,71.75 60.64,71.75 60.01,71.12 v58.74,71.12
INNER_SUPPLY_BUS0
  Top 0.254: SUPPLY.1 90.17,5.08 91.44,6.35 91.44,14.61 92.08,15.24 U2.13
INNER_SUPPLY_BUS1  (via drill 0.35)
  Top 0.254: v94.93,13.34 94.93,14.92 94.61,15.24 U2.15
  Bottom 0.254: v94.93,13.34 89.22,7.62 SUPPLY.2
INNER_SUPPLY_BUS2
  Top 0.254: SUPPLY.3 85.09,1.91 88.58,1.91 96.52,9.84 96.52,19.37 95.89,20 U2.1
INNER_SUPPLY_BUS3
  Top 0.254: SUPPLY.4 86.36,6.35 86.36,2.54 88.58,2.54 93.98,7.94 93.98,19.37 94.61,20 U2.2
INNER_SUPPLY_BUS4
  Top 0.254: SUPPLY.5 82.55,2.22 78.74,2.22 76.2,4.76 76.2,14.61 75.56,15.24 U1.13
INNER_SUPPLY_BUS5
  Top 0.254: SUPPLY.6 82.55,21.59 77.47,21.59 77.47,16.19 78.11,15.56 U1.15
INNER_SUPPLY_BUS6
  Top 0.254: SUPPLY.7 81.28,6.35 81.28,18.1 79.38,20 U1.1
INNER_SUPPLY_BUS7
  Top 0.254: SUPPLY.8 78.74,8.89 78.74,19.37 78.11,20 U1.2
INNER_SUPPLY_BUS8  (via drill 0.35)
  Top 0.254: v59.37,9.53 59.37,14.92 59.05,15.24 U3.13
  Bottom 0.254: v59.37,9.53 60.01,8.89 72.71,8.89 73.66,7.94 73.66,6.99 73.98,6.99 74.61,6.35 76.2,6.35 SUPPLY.9
INNER_SUPPLY_BUS9  (via drill 0.35)
  Top 0.254: v61.59,11.43 U3.15
  Bottom 0.254: v61.59,11.43 61.91,11.75 70.17,11.75 71.75,10.16 74.93,10.16 SUPPLY.10
INNER_SUPPLY_BUS10  (via drill 0.35)
  Top 0.254: v63.5,6.99 63.5,7.94 64.14,8.57 64.14,18.73 62.87,20 U3.1
  Bottom 0.254: v63.5,6.99 64.14,6.35 73.66,6.35 SUPPLY.11
INNER_SUPPLY_BUS11  (via drill 0.35)
  Top 0.254: U3.2 61.59,18.1 60.33,16.83 58.42,16.83 58.42,7.3 59.37,6.35 60.96,6.35 60.96,8.57 v63.18,10.79
  Bottom 0.254: v63.18,10.79 70.48,10.79 71.75,9.53 73.03,9.53 SUPPLY.12
INNER_SUPPLY_BUS12  (via drill 0.35)
  Top 0.254: v47.62,15.24 47.62,13.97 45.72,13.97 45.72,16.83 43.18,16.83 43.18,16.19 42.55,15.56 U4.13 | SUPPLY.13 v72.39,2.22
  Bottom 0.254: v47.62,15.24 47.94,15.56 68.9,15.56 69.85,14.61 94.61,14.61 95.89,13.34 95.89,8.57 93.66,8.57 87.31,2.22 v72.39,2.22
INNER_SUPPLY_BUS13  (via drill 0.35)
  Top 0.254: U4.15 45.09,12.38 47.62,9.84 47.62,8.57 48.26,7.94 48.26,4.45 v50.48,2.22 | v68.58,2.22 71.12,4.76 71.12,5.71 72.39,6.99 SUPPLY.14
  Bottom 0.254: v50.48,2.22 51.44,1.27 67.63,1.27 v68.58,2.22
INNER_SUPPLY_BUS14  (via drill 0.35)
  Top 0.254: v49.53,27.62 49.53,23.5 46.35,20.32 U4.1 | v66.99,27.3 68.58,25.72 68.58,16.51 68.26,16.19 v68.26,14.61 | v70.48,13.65 70.8,13.34 70.8,8.26 71.12,7.94 71.12,6.35 SUPPLY.15
  Bottom 0.254: v49.53,27.62 49.85,27.94 66.36,27.94 v66.99,27.3 | v68.26,14.61 69.22,13.65 v70.48,13.65
INNER_SUPPLY_BUS15  (via drill 0.35)
  Top 0.254: v47.62,16.19 47.62,16.83 45.72,18.73 45.72,19.37 45.09,20 U4.2 | v69.22,16.19 69.53,15.88 69.53,7.94 SUPPLY.16
  Bottom 0.254: v69.22,16.19 v47.62,16.19
INNER_SUPPLY_BUS16  (via drill 0.35)
  Top 0.254: v24.13,21.91 24.13,18.73 25.4,17.46 25.4,16.19 26.04,15.56 U5.13 | v67.63,19.05 67.31,18.73 67.31,9.21 68.58,7.94 68.58,6.35 SUPPLY.17
  Bottom 0.254: v24.13,21.91 26.99,19.05 48.9,19.05 49.21,18.73 53.66,18.73 53.98,19.05 v67.63,19.05
INNER_SUPPLY_BUS17  (via drill 0.35)
  Top 0.254: v28.26,23.81 27.94,23.5 27.94,18.73 28.57,18.73 30.48,16.83 30.48,13.97 29.21,13.97 29.21,14.61 28.57,15.24 U5.15 | v66.99,23.5 66.67,23.18 66.67,8.26 SUPPLY.18
  Bottom 0.254: v28.26,23.81 28.57,23.5 v66.99,23.5
INNER_SUPPLY_BUS18  (via drill 0.35)
  Top 0.254: v34.61,2.22 33.02,3.81 33.02,16.83 29.84,20 U5.1 | v49.53,2.22 50.48,1.27 58.1,1.27 v58.1,4.13
  Bottom 0.254: v49.53,2.22 v34.61,2.22 | v58.1,4.13 58.42,3.81 62.55,3.81 63.82,5.08 SUPPLY.19
INNER_SUPPLY_BUS19  (via drill 0.35)
  Top 0.254: v29.21,24.45 29.21,20.95 28.57,20.32 U5.2 | v75.25,22.86 76.2,21.91 76.2,18.1 74.93,16.83 74.93,9.21 73.66,7.94 73.66,2.54 72.39,1.27 63.5,1.27 63.5,6.03 64.77,7.3 SUPPLY.20
  Bottom 0.254: v29.21,24.45 73.66,24.45 v75.25,22.86
INNER_SUPPLY_BUS20  (via drill 0.35)
  Top 0.254: v8.57,21.91 8.89,21.59 8.89,16.19 9.53,15.56 U6.13 | v48.26,20 48.9,20.64 50.16,20.64 50.16,11.75 v49.85,11.43 | v53.66,11.11 55.88,8.89 55.88,7.3 56.83,6.35 58.42,6.35 58.42,4.76 59.37,3.81 62.23,3.81 SUPPLY.21
  Bottom 0.254: v8.57,21.91 9.53,22.86 33.66,22.86 36.51,20 v48.26,20 | v49.85,11.43 50.16,11.11 v53.66,11.11
INNER_SUPPLY_BUS21  (via drill 0.35)
  Top 0.254: v11.75,17.14 11.75,15.88 12.06,15.56 U6.15 | v65.09,9.84 v65.09,14.61 | v63.18,9.84 62.23,8.89 SUPPLY.22
  Bottom 0.254: v11.75,17.14 14.29,14.61 47.31,14.61 47.62,14.29 53.66,14.29 53.98,14.61 v65.09,14.61 | v63.18,9.84 v65.09,9.84
INNER_SUPPLY_BUS22  (via drill 0.35)
  Top 0.254: v12.7,4.45 12.7,19.37 13.34,20 U6.1
  Bottom 0.254: v12.7,4.45 14.29,2.86 34.29,2.86 34.61,3.17 51.75,3.17 53.34,4.76 53.34,5.4 54.29,6.35 58.42,6.35 SUPPLY.23
INNER_SUPPLY_BUS23  (via drill 0.35)
  Top 0.254: v12.7,28.89 12.7,20.95 12.06,20.32 U6.2 | v61.28,30.48 62.23,29.53 62.23,11.75 62.55,11.43 62.55,11.11 59.69,8.26 SUPPLY.24
  Bottom 0.254: v12.7,28.89 14.29,30.48 v61.28,30.48
N$1  (via drill 0.35)
  Top 0.61: 88.27,20.32 87,20.32 U2.8 87,20 v85.72,20 85.41,20.32 85.41,78.11 84.45,79.06 84.45,83.82 v84.14,84.14 | 88.27,20.32 89.53,20.32 U2.6 | 88.27,20.32 U2.7 | 71.75,20.32 70.48,20.32 U1.8 v70.48,18.1 | 71.75,20.32 73.03,20.32 U1.6 | 71.75,20.32 U1.7 | 55.24,20.32 53.98,20.32 U3.8 v53.98,18.1 | 55.24,20.32 56.52,20.32 U3.6 | 55.24,20.32 U3.7 | 38.73,20.32 37.47,20.32 U4.8 v37.47,18.1 | 38.73,20.32 40.01,20.32 U4.6 | 38.73,20.32 U4.7 | 5.71,20.32 4.45,20.32 U6.8 | 5.71,20.32 6.99,20.32 | 5.71,20.32 U6.7 | 22.23,20.32 20.95,20.32 U5.8 20.95,20 v20,20.95 | 22.23,20.32 23.5,20.32 U5.6 | 22.23,20.32 U5.7 | 6.99,20.32 7.3,20.64 v7.3,21.91 | 6.99,20.32 U6.6
  Bottom 0.61: 78.11,85.09 76.83,85.09 | 78.11,85.09 79.38,85.09 | 78.11,85.09 U8.7 | 94.61,85.09 93.34,85.09 U7.6 | 94.61,85.09 95.89,85.09 U7.8 | 79.38,85.09 81.92,87.63 84.14,87.63 | 84.14,87.63 92.08,87.63 94.61,85.09 | 79.38,85.09 U8.8 | 94.61,85.09 U7.7 | 61.59,85.09 60.33,85.09 | 61.59,85.09 62.55,85.09 | 62.55,85.09 62.87,85.09 U9.8 | 61.59,85.09 U9.7 | 45.09,85.09 43.81,85.09 | 45.09,85.09 46.35,85.09 U10.8 | 45.09,85.09 U10.7 | 12.06,85.09 10.79,85.09 U12.6 | 12.06,85.09 13.34,85.09 | 12.06,85.09 U12.7 | 28.57,85.09 27.94,85.09 | 27.94,85.09 27.3,85.09 U11.6 | 28.57,85.09 29.84,85.09 | 28.57,85.09 U11.7 | 13.34,85.09 15.24,87 26.04,87 27.94,85.09 | 13.34,85.09 U12.8 | 43.81,87.63 43.81,85.09 | 43.81,87.63 32.38,87.63 29.84,85.09 | 43.81,85.09 U10.6 | 29.84,85.09 U11.8 | 60.33,85.09 60.33,87.63 43.81,87.63 | 60.33,85.09 U9.6 | 76.83,85.09 76.83,87.63 65.09,87.63 62.55,85.09 | 76.83,85.09 U8.6 | v85.72,20 83.82,18.1 v70.48,18.1 v53.98,18.1 v37.47,18.1 37.15,18.41 22.54,18.41 v20,20.95 8.26,20.95 v7.3,21.91 8.89,23.5 11.75,23.5 13.02,24.77 28.26,24.77 28.89,25.4 29.53,25.4 29.84,25.08 41.59,25.08 B1.GND@2 | v84.14,84.14 84.14,87.63
N$2
  Top 0.254: U13.2 87.63,50.16 87,50.8 87,52.07 90.17,52.07 90.49,51.75 90.49,48.9 U13.6 93.98,48.9 94.61,48.26 94.61,46.99 93.98,46.35 93.98,20.95 93.34,20.32 U2.3
N$3  (via drill 0.35)
  Top 0.61: U13.5 89.85,47.62 | 89.85,47.62 U13.4 v86.36,47.62 | U13.1 89.85,51.44 89.85,47.62 | U14.5 73.34,47.62 | 73.34,47.62 U14.4 v70.17,47.62 | U14.1 73.34,51.44 73.34,47.62 | U15.5 56.83,47.62 | 56.83,47.62 U15.4 v53.66,47.62 | U15.1 56.83,51.44 56.83,47.62 | U16.5 40.32,47.62 | 40.32,47.62 U16.4 v33.97,47.62 | U16.1 40.32,51.44 40.32,47.62 | 7.3,47.62 U18.5 16.83,47.62 v16.83,47.31 | 7.3,47.62 U18.4 | U18.1 7.3,51.44 7.3,47.62 | U17.5 23.81,47.62 | 23.81,47.62 U17.4 22.23,47.62 22.23,47.31 v20.64,47.31 | 23.81,51.44 U17.1 | 23.81,47.62 23.81,51.44 | B1.GND@1 26.04,74.3 26.04,53.66 23.81,51.44
  Bottom 0.61: v16.83,47.31 v20.64,47.31 33.66,47.31 v33.97,47.62 v53.66,47.62 v70.17,47.62 v86.36,47.62
N$4  (via drill 0.35)
  Top 0.61: v15.56,15.56 13.34,15.56 U6.16 | v28.89,17.14 29.84,16.19 U5.16 | v46.35,17.14 U4.16 | v63.18,17.14 63.18,15.88 62.87,15.56 U3.16 | v79.69,17.14 79.69,15.88 79.38,15.56 U1.16 | v95.57,17.14 95.57,15.88 95.89,15.56 U2.16 | v20,77.47 v20,79.38 | v29.84,76.83 v32.07,79.06 | U18.7 8.57,50.16 8.57,70.48 4.45,74.61 v4.45,78.42 | v30.8,50.16 U17.7 | U16.7 42.23,50.16 | U15.7 57.78,50.16 57.78,51.75 57.31,52.23 | 57.31,52.23 57.15,52.39 48.26,52.39 | 48.26,52.39 42.23,52.39 42.23,50.16 | 42.23,50.16 v41.91,50.16 | U14.7 74.3,50.16 74.3,51.75 73.82,52.23 | 73.82,52.23 73.66,52.39 63.82,52.39 | 63.82,52.39 57.47,52.39 57.31,52.23 | v91.44,50.16 U13.7 | 48.26,52.39 48.26,77.47 | 48.26,77.47 v48.26,80.01 | v64.77,79.06 63.82,78.11 63.82,52.39 | v81.6,79.06 80.96,78.42 80.96,59.37 73.82,52.23 | 48.26,77.47 v47.94,77.47
  Bottom 0.61: v15.56,15.56 17.14,17.14 v28.89,17.14 v46.35,17.14 v63.18,17.14 v79.69,17.14 93.66,17.14 | 93.66,17.14 v95.57,17.14 | v20,79.38 20.32,79.38 20.95,80.01 U11.16 | 21.11,76.36 22.54,74.93 B1.VIN | 21.11,76.36 v20,77.47 5.4,77.47 v4.45,78.42 U12.16 | v32.07,79.06 36.51,79.06 37.47,80.01 U10.16 | 21.11,76.36 21.27,76.52 29.53,76.52 v29.84,76.83 30.48,77.47 v47.94,77.47 | v30.8,50.16 v41.91,50.16 v91.44,50.16 93.66,50.16 93.66,17.14 | v48.26,80.01 53.98,80.01 U9.16 | v64.77,79.06 69.53,79.06 70.48,80.01 U8.16 | v81.6,79.06 86.04,79.06 87,80.01 U7.16
N$5  (via drill 0.35)
  Top 0.61: v4.13,48.9 U18.3 | v20.64,48.26 21.27,48.9 U17.3 | v33.97,48.9 U16.3 | v53.66,48.9 U15.3 | v70.17,48.9 U14.3 | v86.36,48.9 U13.3 | v31.75,48.26 B1.5V
  Bottom 0.61: v4.13,48.9 4.76,48.26 v20.64,48.26 v31.75,48.26 33.34,48.26 v33.97,48.9 v53.66,48.9 v70.17,48.9 v86.36,48.9
N$6  (via drill 0.35)
  Top 0.254: v83.5,19.05 87,15.56 U2.9 | U1.9 70.48,15.56 70.17,15.88 70.17,17.46 69.53,18.1 v69.53,19.05 69.22,19.37 69.22,26.04 v66.99,28.26 | v4.45,18.41 U6.9 | B1.D4 16.51,15.56 20.95,15.56 U5.9 | v37.47,11.75 v37.47,13.65 U4.9 | v53.98,13.65 U3.9
  Bottom 0.254: v83.5,19.05 v69.53,19.05 | v37.47,11.75 37.15,12.06 11.11,12.06 5.71,17.46 5.4,17.46 v4.45,18.41 4.45,27.94 15.24,27.94 B1.D4 17.78,25.4 24.77,25.4 27.94,28.57 66.67,28.57 v66.99,28.26 | v37.47,13.65 v53.98,13.65
N$7
  Top 0.254: U14.6 78.11,48.9 78.11,46.99 77.79,46.67 76.83,46.67 | 76.83,46.67 69.22,46.67 69.22,48.9 70.48,50.16 U14.2 | 76.83,46.67 U1.3
N$8  (via drill 0.35)
  Top 0.254: v5.4,18.41 5.4,15.88 5.71,15.56 U6.10 | B1.D3 13.97,27.94 17.14,27.94 17.78,27.3 17.78,17.46 20.95,17.46 21.59,16.83 21.59,16.19 22.23,15.56 U5.10 | v38.42,12.7 38.42,14.92 38.73,15.24 U4.10 | v54.93,11.75 54.93,14.92 55.24,15.24 U3.10 | v71.75,11.75 U1.10 | v87.63,12.7 87.63,14.61 88.27,15.24 U2.10
  Bottom 0.254: B1.D3 12.06,24.77 5.4,24.77 v5.4,18.41 11.11,12.7 v38.42,12.7 39.37,11.75 39.69,11.75 40.32,12.38 49.85,12.38 50.16,12.06 54.61,12.06 v54.93,11.75 55.56,12.38 70.17,12.38 70.48,12.06 71.44,12.06 v71.75,11.75 86.68,11.75 v87.63,12.7
N$9  (via drill 0.35)
  Top 0.254: v56.2,13.65 56.2,14.92 56.52,15.24 U3.11 | v72.71,12.7 73.03,13.02 U1.11 | v88.9,13.65 88.9,14.61 89.53,15.24 U2.11 | 10.16,10.48 8.89,10.48 7.62,11.75 7.62,14.61 6.99,15.24 U6.11 | 10.16,10.48 10.16,17.46 11.43,18.73 B1.D2 | 15.88,1.27 23.18,8.57 23.18,14.92 23.5,15.24 U5.11 | 15.88,1.27 10.16,1.27 10.16,10.48 | 15.88,1.27 34.61,1.27 38.1,4.76 38.1,7.94 39.69,9.53 v39.69,12.7 39.69,14.92 40.01,15.24 U4.11
  Bottom 0.254: v88.9,13.65 73.66,13.65 v72.71,12.7 70.48,12.7 70.17,13.02 56.83,13.02 v56.2,13.65 55.24,12.7 50.16,12.7 49.85,13.02 40.01,13.02 v39.69,12.7
N$10
  Top 0.254: U15.6 61.59,48.9 61.59,46.99 61.28,46.67 60.33,46.67 | 60.33,46.67 52.7,46.67 52.7,48.9 53.98,50.16 U15.2 | 60.33,46.67 U3.3
N$11  (via drill 0.35)
  Top 0.254: v16.83,80.33 17.78,79.38 17.78,68.26 | 17.78,68.26 17.78,27.94 B1.D5 | v59.05,81.92 v59.05,74.3 | 17.78,68.26 22.86,68.26 22.86,79.69 26.04,82.87 27.3,82.87 v27.3,81.92
  Bottom 0.254: U12.11 10.79,82.23 14.92,82.23 v16.83,80.33 | U8.11 76.83,82.23 80.33,82.23 80.64,81.92 85.41,81.92 85.72,82.23 92.08,82.23 93.34,80.96 | 93.34,80.96 U7.11 93.34,80.33 | U11.11 v27.3,81.92 27.3,82.23 30.8,82.23 31.11,81.92 37.78,81.92 38.73,82.87 40.64,82.87 41.27,82.23 | 41.27,82.23 41.91,81.6 43.18,81.6 43.81,80.96 U10.11 | U9.11 60.33,82.23 59.05,82.23 | 59.05,82.23 57.47,82.23 56.52,83.19 56.2,83.19 55.24,82.23 47.94,82.23 47.62,81.92 47.31,82.23 41.27,82.23 | 93.34,80.96 93.98,81.6 96.52,81.6 96.52,75.88 71.44,75.88 69.53,73.98 69.22,74.3 v59.05,74.3 | 59.05,82.23 v59.05,81.92
N$12  (via drill 0.35)
  Top 0.254: B1.D6 19.05,29.21 19.05,63.82 25.4,70.17 v25.4,77.79
  Bottom 0.254: U12.10 12.06,78.11 19.68,78.11 20,78.42 24.45,78.42 24.77,78.11 25.4,78.11 | 27.94,78.11 25.4,78.11 | 27.94,78.11 28.57,78.74 U11.10 | 45.09,78.11 U10.10 | 27.94,78.11 45.09,78.11 | 61.59,78.11 U9.10 | 61.59,78.11 48.26,78.11 47.94,78.42 47.62,78.42 47.31,78.11 45.09,78.11 | 78.11,78.11 U8.10 | 61.59,78.11 78.11,78.11 | U7.10 94.61,77.47 84.45,77.47 84.14,77.15 80.64,77.15 79.69,78.11 78.11,78.11 | 25.4,78.11 v25.4,77.79
N$13
  Top 0.254: U16.2 38.1,50.16 37.47,50.8 37.47,52.07 40.64,52.07 40.96,51.75 40.96,48.9 U16.6 44.45,48.9 45.09,48.26 45.09,46.99 44.45,46.35 44.45,20.95 43.81,20.32 U4.3
N$14  (via drill 0.35)
  Top 0.254: v69.22,80.01 69.53,79.69 v69.53,77.15 | v80.33,79.06 80.01,78.74 v80.01,76.83 | v24.13,90.49 v14.92,81.28 | v29.84,90.81 32.07,88.58 v32.07,80.96 33.02,80.01 33.02,66.04 | v47.31,79.06 46.67,78.42 46.67,76.52 | 46.67,76.52 46.67,68.58 44.13,66.04 33.02,66.04 | v26.99,29.53 33.02,35.56 33.02,66.04 | 46.67,76.52 v46.99,76.52
  Bottom 0.254: v69.22,80.01 62.87,80.01 U9.9 | 80.01,76.52 94.3,76.52 95.89,78.11 U7.9 | 80.01,76.52 70.17,76.52 v69.53,77.15 69.22,76.83 48.26,76.83 47.94,76.52 v46.99,76.52 | v80.33,79.06 79.38,80.01 U8.9 | 80.01,76.52 v80.01,76.83 | v14.92,81.28 14.29,81.28 13.34,80.33 U12.9 | v24.13,90.49 24.45,90.81 v29.84,90.81 | v32.07,80.96 31.43,80.33 29.84,80.33 U11.9 | v47.31,79.06 46.35,80.01 U10.9 | v26.99,29.53 B1.D7
N$15  (via drill 0.35)
  Top 0.254: B1.A0 19.05,81.28 16.83,81.28 15.88,80.33 14.92,80.33 13.97,81.28 13.97,82.23 13.65,82.55 R1.2 13.34,82.55 v9.21,86.68
  Bottom 0.254: U12.3 6.99,86.68 v9.21,86.68
N$16
  Top 0.254: U17.6 28.57,48.9 28.57,46.99 27.94,46.35 26.04,46.35 | 26.04,46.35 19.68,46.35 19.68,48.26 21.59,50.16 U17.2 | 26.04,46.35 26.04,29.53 26.67,28.89 26.67,20.95 27.3,20.32 U5.3
N$17  (via drill 0.35)
  Top 0.254: R2.2 31.11,82.55 v31.11,82.87 | B1.A1 16.83,75.25 v16.83,79.06
  Bottom 0.254: v31.11,82.87 24.77,82.87 23.81,83.82 | 23.81,83.82 23.5,84.14 U11.3 | v16.83,79.06 20,82.23 22.23,82.23 23.81,83.82
N$18  (via drill 0.35)
  Top 0.254: v64.14,82.87 64.14,82.55 R4.2 62.87,82.55 62.55,82.23 62.55,68.9 v60.64,66.99
  Bottom 0.254: v64.14,82.87 57.78,82.87 56.52,84.14 U9.3 | B1.A3 18.1,68.26 43.81,68.26 44.13,68.58 48.26,68.58 49.85,66.99 v60.64,66.99
N$19
  Top 0.254: U18.6 7.94,48.9 7.94,51.75 7.62,52.07 4.45,52.07 4.45,50.8 4.76,50.48 | 4.76,50.48 5.08,50.16 U18.2 | 4.76,50.48 3.17,48.9 3.17,48.26 10.16,41.27 10.16,20.95 10.79,20.32 U6.3
N$20  (via drill 0.35)
  Top 0.254: v80.64,82.87 80.64,82.55 R5.2 79.38,82.55 79.06,82.23 79.06,66.04 73.66,66.04 73.34,66.36 v72.07,66.36
  Bottom 0.254: v80.64,82.87 74.3,82.87 73.03,84.14 U8.3 | B1.A4 8.89,67.63 43.81,67.63 44.13,67.94 46.35,67.94 48.26,66.04 71.75,66.04 v72.07,66.36
N$21  (via drill 0.35)
  Top 0.61: v15.88,76.52 12.38,80.01 12.38,82.23 12.06,82.55 R1.1 | 28.73,82.39 28.89,82.23 28.89,75.25 B1.GND@0 | 28.73,82.39 28.57,82.55 R2.1 | v45.09,88.58 45.09,82.55 R3.1 | v31.11,88.58 28.89,86.36 28.89,82.55 28.73,82.39 | v61.59,87.63 61.59,82.55 R4.1 | v78.11,87.63 78.11,82.55 R5.1 | v93.66,87.31 93.66,83.19 94.3,82.55 R6.1
  Bottom 0.61: v15.88,76.52 19.68,76.52 22.86,73.34 27.62,73.34 B1.GND@0 | v31.11,88.58 v45.09,88.58 60.64,88.58 60.8,88.42 | 60.8,88.42 v61.59,87.63 | 77.31,88.42 77.15,88.58 60.96,88.58 60.8,88.42 | 77.31,88.42 v78.11,87.63 | v93.66,87.31 92.39,88.58 77.47,88.58 77.31,88.42
N$22  (via drill 0.35)
  Top 0.254: v97.16,82.55 R6.2 95.89,82.55 95.89,79.69 v86.36,70.17 | B1.A5 11.75,69.53 v11.75,64.14
  Bottom 0.254: v97.16,82.55 96.84,82.87 90.17,82.87 89.53,83.5 U7.3 | v11.75,64.14 14.92,60.96 77.15,60.96 v86.36,70.17
N$23  (via drill 0.35)
  Top 0.254: v47.62,82.87 47.62,82.55 R3.2 46.35,82.55 46.04,82.23 46.04,73.03 v45.72,72.71
  Bottom 0.254: v47.62,82.87 41.27,82.87 40.01,84.14 U10.3 | B1.A2 16.19,72.71 v45.72,72.71
OUTER_SENSE_BUS0  (via drill 0.35)
  Top 0.254: v68.26,64.45 71.12,67.31 v71.12,96.52 | v57.47,97.79 58.1,97.79 58.42,98.11 59.69,98.11 SENSE.27
  Bottom 0.254: U12.14 6.99,78.74 5.08,78.74 5.08,81.6 3.81,81.6 3.49,81.28 3.49,66.67 43.5,66.67 45.72,64.45 v68.26,64.45 | v71.12,96.52 69.53,98.11 57.78,98.11 v57.47,97.79
OUTER_SENSE_BUS1  (via drill 0.35)
  Top 0.254: v9.84,78.42 12.7,75.56 v12.7,64.14 | v51.44,62.87 60.01,71.44 60.01,92.39 SENSE.28
  Bottom 0.254: U12.12 9.53,78.42 v9.84,78.42 | v12.7,64.14 13.97,62.87 v51.44,62.87
OUTER_SENSE_BUS2  (via drill 0.35)
  Top 0.254: v14.29,83.5 25.4,94.61 25.4,95.57 28.57,98.74 62.23,98.74 SENSE.29
  Bottom 0.254: U12.5 9.53,83.5 v14.29,83.5
OUTER_SENSE_BUS3  (via drill 0.35)
  Top 0.254: v8.26,83.19 15.24,76.2 v15.24,61.91 | v58.1,61.91 63.18,66.99 63.18,80.96 65.09,82.87 65.09,86.04 62.23,88.9 SENSE.30
  Bottom 0.254: v8.26,83.19 U12.4 | v58.1,61.91 v15.24,61.91
OUTER_SENSE_BUS4  (via drill 0.35)
  Top 0.254: v23.5,81.92 21.91,80.33 v21.91,69.22 | v74.61,67.94 74.61,85.72 73.66,86.68 73.66,95.57 71.75,97.47 64.77,97.47 SENSE.31
  Bottom 0.254: v23.5,81.92 U11.14 | v21.91,69.22 48.26,69.22 49.53,67.94 v74.61,67.94
OUTER_SENSE_BUS5  (via drill 0.35)
  Top 0.254: v26.04,81.92 27.94,80.01 v27.94,71.12 | v64.77,70.17 65.72,71.12 65.72,86.04 66.36,86.68 66.36,91.12 SENSE.32
  Bottom 0.254: v26.04,81.92 U11.12 | v27.94,71.12 28.26,70.8 56.52,70.8 57.78,69.53 61.28,69.53 61.91,70.17 v64.77,70.17
OUTER_SENSE_BUS6  (via drill 0.35)
  Top 0.254: v33.97,86.68 35.56,88.27 v35.56,95.89
  Bottom 0.254: U11.5 26.04,83.5 30.8,83.5 v33.97,86.68 | v35.56,95.89 36.2,96.52 58.1,96.52 58.42,96.2 59.05,96.2 59.37,96.52 66.04,96.52 SENSE.33
OUTER_SENSE_BUS7  (via drill 0.35)
  Top 0.254: v20,83.5 20.95,82.55 v20.95,70.17 | v61.59,68.9 60.64,69.85 60.64,92.08 60.96,92.39 60.96,93.03 61.91,93.98 67.31,93.98 SENSE.34
  Bottom 0.254: U11.4 24.77,86.36 21.59,86.36 21.59,83.5 v20,83.5 | v20.95,70.17 47.94,70.17 49.21,68.9 v61.59,68.9
OUTER_SENSE_BUS8  (via drill 0.35)
  Top 0.254: v39.69,81.92 42.86,78.74 v42.86,76.52 | v66.67,72.71 66.67,86.36 66.99,86.68 66.99,90.81 68.58,92.39 68.58,93.98 SENSE.35
  Bottom 0.254: U10.14 40.01,81.6 v39.69,81.92 | v42.86,76.52 46.67,72.71 60.33,72.71 60.64,73.03 66.36,73.03 v66.67,72.71
OUTER_SENSE_BUS9  (via drill 0.35)
  Top 0.254: v50.16,80.96 50.48,80.64 v50.48,75.25 | v69.53,74.93 70.48,75.88 70.48,92.08 SENSE.36
  Bottom 0.254: U10.12 42.55,78.74 44.45,78.74 44.45,81.6 47.31,81.6 47.94,80.96 v50.16,80.96 | v50.48,75.25 67.94,75.25 68.26,74.93 v69.53,74.93
OUTER_SENSE_BUS10  (via drill 0.35)
  Top 0.254: v56.83,86.68 58.1,87.95 58.1,92.08 58.42,92.39 v58.42,97.16
  Bottom 0.254: U10.5 42.55,83.5 47.31,83.5 47.62,83.82 53.02,83.82 53.34,83.5 55.88,83.5 55.88,86.68 v56.83,86.68 | v58.42,97.16 69.53,97.16 71.44,95.25 SENSE.37
OUTER_SENSE_BUS11  (via drill 0.35)
  Top 0.254: v41.59,86.68 43.5,84.77 43.5,76.83 v43.81,76.52 | v72.07,73.34 72.39,73.66 SENSE.38
  Bottom 0.254: U10.4 41.27,86.68 v41.59,86.68 | v43.81,76.52 46.99,73.34 60.33,73.34 60.64,73.66 69.22,73.66 69.53,73.34 v72.07,73.34
OUTER_SENSE_BUS12  (via drill 0.35)
  Top 0.254: v56.52,82.23 55.88,82.87 v55.88,97.47
  Bottom 0.254: v56.52,82.23 U9.14 | v55.88,97.47 57.15,98.74 74.61,98.74 76.2,97.16 76.2,95.89 75.56,95.89 SENSE.39
OUTER_SENSE_BUS13  (via drill 0.35)
  Top 0.254: v68.26,81.92 68.9,82.55 v68.9,91.76
  Bottom 0.254: U9.12 59.05,78.74 60.96,78.74 60.96,81.92 v68.26,81.92 | v68.9,91.76 69.22,91.44 73.66,91.44 SENSE.40
OUTER_SENSE_BUS14  (via drill 0.35)
  Top 0.254: v59.05,91.44 v59.05,86.68
  Bottom 0.254: v59.05,86.68 U9.5 | v59.05,91.44 59.37,91.12 68.58,91.12 68.9,90.81 74.61,90.81 76.2,92.39 76.2,95.25 SENSE.41
OUTER_SENSE_BUS15  (via drill 0.35)
  Top 0.254: v74.61,86.68 75.56,85.72 76.52,85.72 76.52,91.76 SENSE.42
  Bottom 0.254: U9.4 57.78,83.5 63.82,83.5 64.14,83.82 66.67,83.82 67.63,82.87 71.75,82.87 72.39,83.5 72.39,86.68 v74.61,86.68
OUTER_SENSE_BUS16  (via drill 0.35)
  Top 0.254: v80.33,81.28 81.6,82.55 81.6,92.08 81.28,92.39 81.28,93.98 SENSE.43
  Bottom 0.254: U8.14 73.03,78.74 77.47,78.74 77.47,81.6 80.01,81.6 v80.33,81.28
OUTER_SENSE_BUS17  (via drill 0.35)
  Top 0.254: v75.56,81.92 77.15,83.5 77.15,89.85 SENSE.44
  Bottom 0.254: v75.56,81.92 U8.12
OUTER_SENSE_BUS18  (via drill 0.35)
  Top 0.254: v75.56,86.68 75.88,87 75.88,92.08 76.2,92.39 76.2,95.57 77.15,96.52 82.55,96.52 SENSE.45
  Bottom 0.254: v75.56,86.68 U8.5
OUTER_SENSE_BUS19  (via drill 0.35)
  Top 0.254: SENSE.46 v82.55,86.04
  Bottom 0.254: U8.4 74.3,83.5 80.01,83.5 v82.55,86.04
OUTER_SENSE_BUS20  (via drill 0.35)
  Top 0.254: v89.53,78.42 86.36,81.6 86.36,93.98 SENSE.47
  Bottom 0.254: v89.53,78.42 U7.14
OUTER_SENSE_BUS21  (via drill 0.35)
  Top 0.254: v85.72,81.28 85.09,81.92 SENSE.48
  Bottom 0.254: U7.12 92.08,81.6 86.04,81.6 v85.72,81.28
OUTER_SENSE_BUS22  (via drill 0.35)
  Top 0.254: v91.76,86.68 88.9,89.53 88.9,93.98 SENSE.49
  Bottom 0.254: U7.5 92.08,86.68 v91.76,86.68
OUTER_SENSE_BUS23  (via drill 0.35)
  Top 0.254: v90.81,86.68 87.63,89.85 SENSE.50
  Bottom 0.254: v90.81,86.68 U7.4
OUTER_SUPPLY_BUS0  (via drill 0.35)
  Top 0.254: v92.71,18.1 92.71,16.19 93.34,15.56 U2.14 | v55.88,25.4 52.7,22.23 52.7,9.53 53.34,8.89 53.34,6.35 SUPPLY.27
  Bottom 0.254: v92.71,18.1 85.72,25.08 56.2,25.08 v55.88,25.4
OUTER_SUPPLY_BUS1  (via drill 0.35)
  Top 0.254: v90.17,6.03 90.17,14.61 90.81,15.24 U2.12 | v57.15,3.49 55.88,4.76 55.88,6.35 SUPPLY.28
  Bottom 0.254: v90.17,6.03 87.95,3.81 79.06,3.81 78.74,4.13 78.11,4.13 77.79,3.81 63.18,3.81 62.55,3.17 57.47,3.17 v57.15,3.49
OUTER_SUPPLY_BUS2  (via drill 0.35)
  Top 0.254: v90.17,21.91 90.17,20.95 90.81,20.32 U2.5 | v56.83,26.04 57.15,25.72 v57.15,9.21
  Bottom 0.254: v90.17,21.91 86.36,25.72 57.15,25.72 v56.83,26.04 | v57.15,9.21 56.83,8.89 54.29,8.89 53.34,7.94 53.34,6.03 53.02,6.03 SUPPLY.29
OUTER_SUPPLY_BUS3  (via drill 0.35)
  Top 0.254: v91.44,21.91 91.44,20.95 92.08,20.32 U2.4 | v53.34,26.99 51.44,25.08 51.44,9.53 51.12,9.21 51.12,8.57 SUPPLY.30
  Bottom 0.254: v91.44,21.91 87,26.35 57.47,26.35 56.83,26.99 v53.34,26.99
OUTER_SUPPLY_BUS4  (via drill 0.35)
  Top 0.254: v78.74,3.17 78.74,7.94 77.47,9.21 77.47,14.61 76.83,15.24 U1.14 | v51.44,2.22 49.53,4.13 SUPPLY.31
  Bottom 0.254: v78.74,3.17 67.31,3.17 66.04,1.91 51.75,1.91 v51.44,2.22
OUTER_SUPPLY_BUS5  (via drill 0.35)
  Top 0.254: v72.71,22.54 73.66,21.59 73.66,16.19 74.3,15.56 U1.12 | v50.48,21.91 50.8,21.59 50.8,9.53 49.53,8.26 SUPPLY.32
  Bottom 0.254: v72.71,22.54 61.59,22.54 61.28,22.86 51.44,22.86 v50.48,21.91
OUTER_SUPPLY_BUS6  (via drill 0.35)
  Top 0.254: U1.5 74.3,21.91 66.99,29.21 66.04,29.21 v66.04,2.86 | v51.12,4.13 v52.39,2.86
  Bottom 0.254: v66.04,2.86 65.72,2.54 52.7,2.54 v52.39,2.86 | v51.12,4.13 50.8,3.81 48.26,3.81 SUPPLY.33
OUTER_SUPPLY_BUS7  (via drill 0.35)
  Top 0.254: v75.25,21.91 75.25,20.64 75.56,20.32 U1.4 | v49.21,19.68 48.58,19.05 v48.58,9.21
  Bottom 0.254: v75.25,21.91 73.34,20 49.53,20 v49.21,19.68 | SUPPLY.34 v48.58,9.21
OUTER_SUPPLY_BUS8  (via drill 0.35)
  Top 0.254: v60.33,11.43 U3.14 | v46.35,10.16 45.72,9.53 45.72,6.35 SUPPLY.35
  Bottom 0.254: v60.33,11.43 59.05,10.16 v46.35,10.16
OUTER_SUPPLY_BUS9  (via drill 0.35)
  Top 0.254: U3.12 57.78,16.83 59.05,18.1 60.96,18.1 60.96,21.59 v61.28,21.91 | v36.51,10.79 v36.51,20.95
  Bottom 0.254: v61.28,21.91 60.33,20.95 v36.51,20.95 | v36.51,10.79 37.78,9.53 42.55,9.53 SUPPLY.36
OUTER_SUPPLY_BUS10  (via drill 0.35)
  Top 0.254: v52.07,9.21 52.07,22.23 54.29,24.45 54.29,26.99 53.34,27.94 53.34,30.48 54.29,30.48 59.69,25.08 59.69,18.73 58.42,18.73 58.42,19.37 57.78,20 U3.5
  Bottom 0.254: v52.07,9.21 50.8,7.94 50.8,6.35 43.18,6.35 SUPPLY.37
OUTER_SUPPLY_BUS11  (via drill 0.35)
  Top 0.254: v54.29,29.53 58.42,25.4 58.42,20.95 59.05,20.32 U3.4 | v36.51,29.53 34.29,27.3 v34.29,9.21
  Bottom 0.254: v36.51,29.53 v54.29,29.53 | v34.29,9.21 35.56,7.94 35.56,6.35 40.64,6.35 SUPPLY.38
OUTER_SUPPLY_BUS12
  Top 0.254: SUPPLY.39 40.64,6.35 40.64,7.94 43.18,10.48 43.18,14.61 43.81,15.24 U4.14
OUTER_SUPPLY_BUS13
  Top 0.254: SUPPLY.40 39.37,8.57 40.64,9.84 40.64,14.61 41.27,15.24 U4.12
OUTER_SUPPLY_BUS14
  Top 0.254: SUPPLY.41 35.56,6.35 35.56,22.86 39.37,22.86 40.64,21.59 40.64,20.95 41.27,20.32 U4.5
OUTER_SUPPLY_BUS15  (via drill 0.35)
  Top 0.254: v40.32,8.57 41.91,10.16 41.91,19.37 42.55,20 U4.4
  Bottom 0.254: v40.32,8.57 40.01,8.89 38.1,8.89 SUPPLY.42
OUTER_SUPPLY_BUS16  (via drill 0.35)
  Top 0.254: v27.3,10.16 U5.14
  Bottom 0.254: v27.3,10.16 28.57,8.89 32.07,8.89 33.02,7.94 33.02,5.08 SUPPLY.43
OUTER_SUPPLY_BUS17  (via drill 0.35)
  Top 0.254: v25.4,10.79 25.4,14.61 24.77,15.24 U5.12
  Bottom 0.254: v25.4,10.79 25.72,11.11 30.8,11.11 SUPPLY.44
OUTER_SUPPLY_BUS18
  Top 0.254: SUPPLY.45 31.75,6.35 28.89,6.35 27.94,7.3 27.94,7.94 26.35,9.53 26.35,10.16 26.67,10.48 26.67,16.83 25.4,18.1 25.4,19.37 24.77,20 U5.5
OUTER_SUPPLY_BUS19
  Top 0.254: U5.4 26.04,18.73 27.94,16.83 27.94,11.43 SUPPLY.46
OUTER_SUPPLY_BUS20  (via drill 0.35)
  Top 0.254: v11.43,6.67 11.43,14.61 10.79,15.24 U6.14
  Bottom 0.254: v11.43,6.67 14.29,3.81 16.19,3.81 16.51,3.49 27.62,3.49 SUPPLY.47
OUTER_SUPPLY_BUS21  (via drill 0.35)
  Top 0.254: v8.89,13.34 8.89,14.61 8.26,15.24 U6.12
  Bottom 0.254: v8.89,13.34 13.02,9.21 27.62,9.21 SUPPLY.48
OUTER_SUPPLY_BUS22  (via drill 0.35)
  Top 0.254: U6.5 8.26,18.73 6.35,16.83 v6.35,12.06
  Bottom 0.254: v6.35,12.06 10.79,7.62 13.02,7.62 16.51,4.13 25.72,4.13 SUPPLY.49
OUTER_SUPPLY_BUS23  (via drill 0.35)
  Top 0.254: U6.4 9.53,22.23 7.62,24.13 3.17,24.13 v3.17,16.19
  Bottom 0.254: v3.17,16.19 10.79,8.57 25.72,8.57 SUPPLY.50

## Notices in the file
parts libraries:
SparkFun-Boards: Licensing: Creative Commons ShareAlike 4.0 International - https://creativecommons.org/licenses/by-sa/4.0
